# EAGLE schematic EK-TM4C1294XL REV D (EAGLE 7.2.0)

## Sheet 1 of 6: TM4C129ENCPDT GPIO
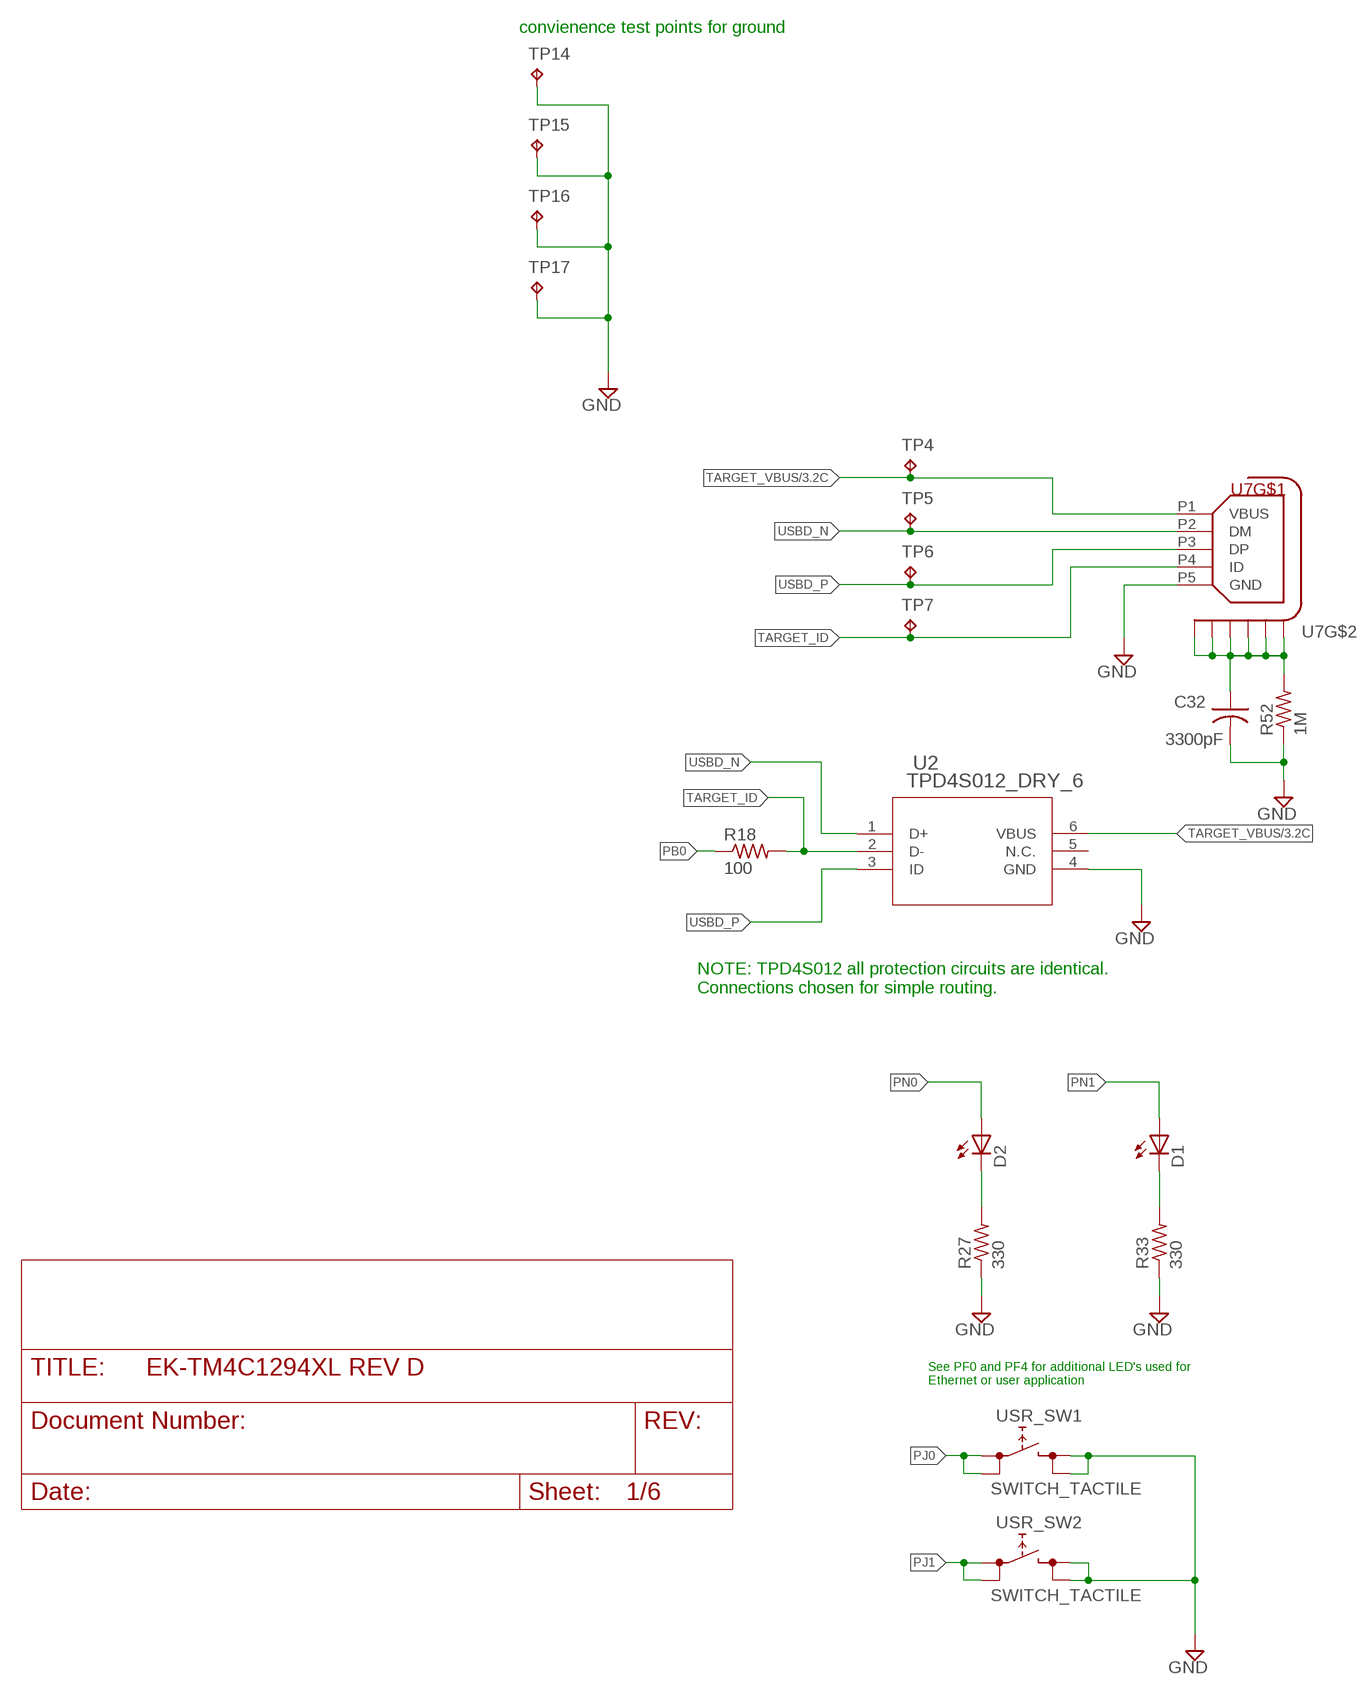
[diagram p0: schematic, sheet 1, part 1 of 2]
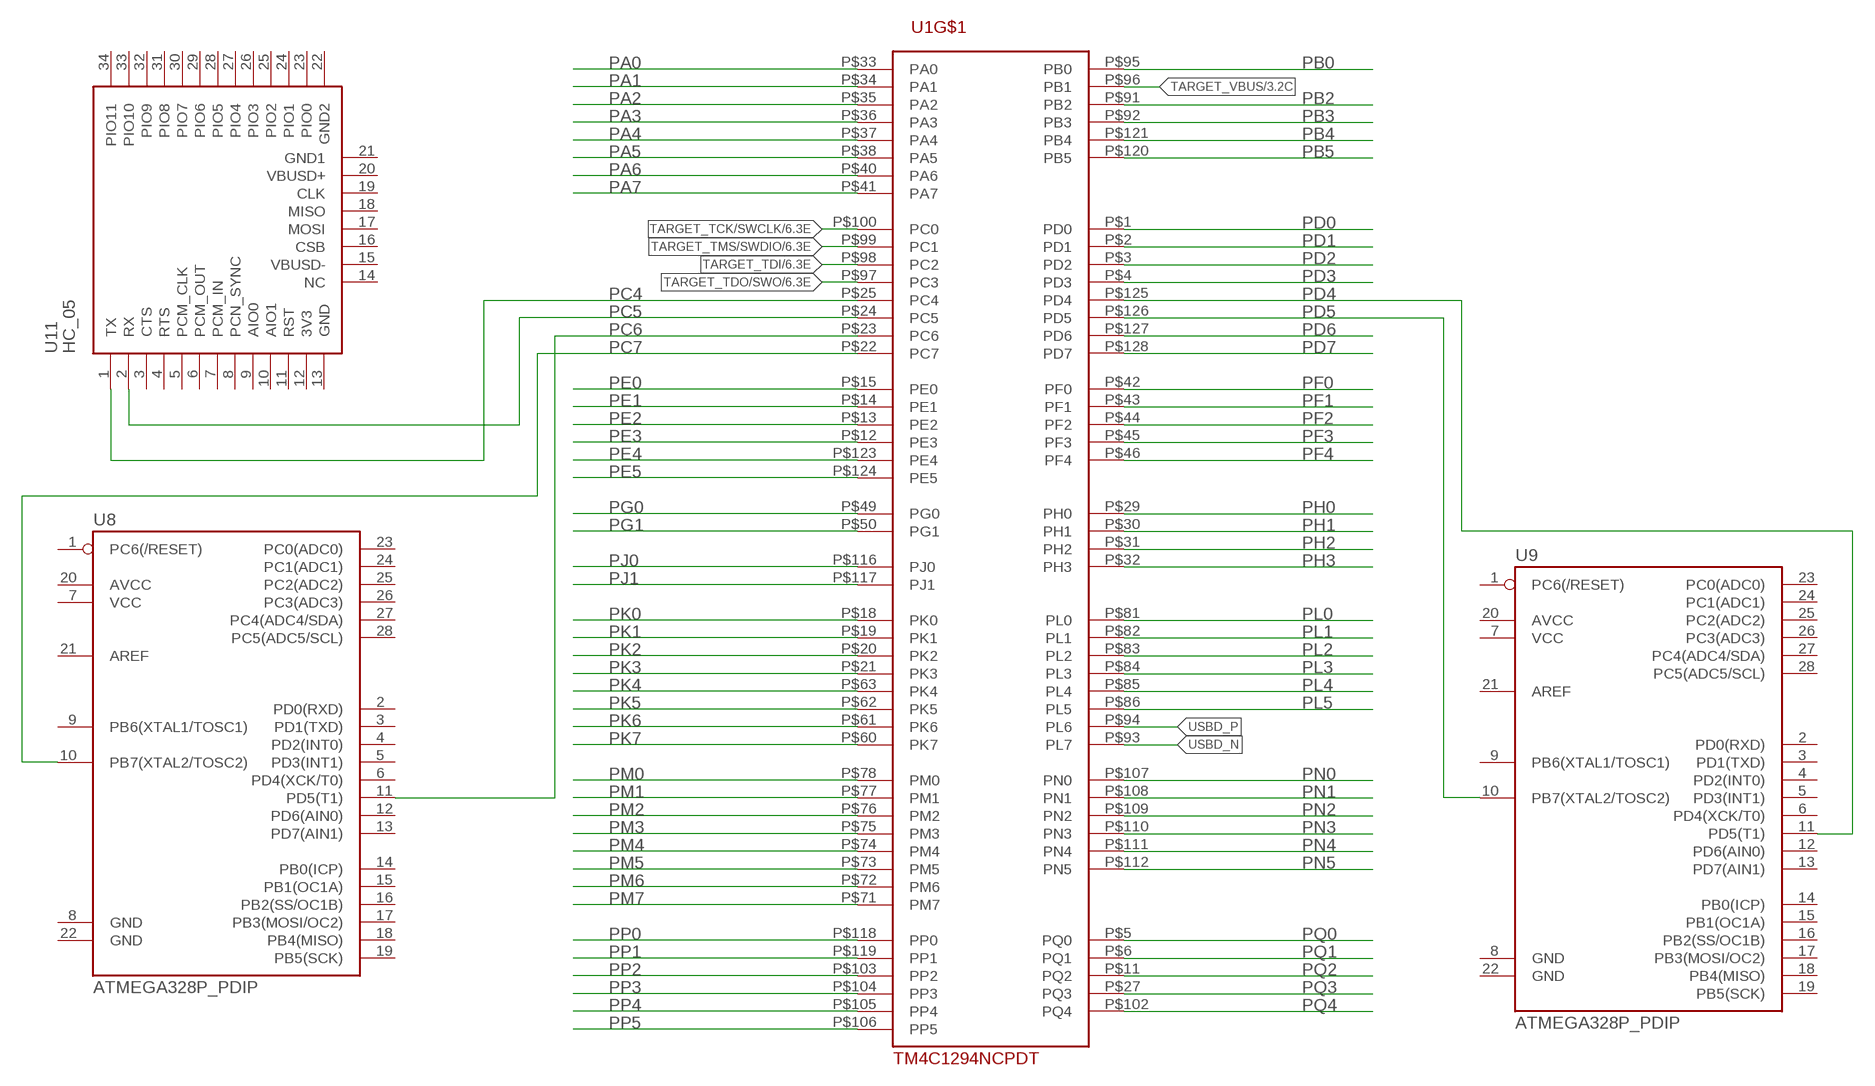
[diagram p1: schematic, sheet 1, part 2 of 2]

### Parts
C32  3300pF  C-USC0603  [C0603]
D1  LEDCHIPLED_0603  [CHIPLED_0603]
D2  LEDCHIPLED_0603  [CHIPLED_0603]
R18  100  R-US_R0402  [R0402]
R27  330  R-US_R0402  [R0402]
R33  330  R-US_R0402  [R0402]
R52  1M  R-US_R0603  [R0603]
TP4  TPPAD1-13  [P1-13]
TP5  TPPAD1-13  [P1-13]
TP6  TPPAD1-13  [P1-13]
TP7  TPPAD1-13  [P1-13]
TP14  TPPAD1-13  [P1-13]
TP15  TPPAD1-13  [P1-13]
TP16  TPPAD1-13  [P1-13]
TP17  TPPAD1-13  [P1-13]
U1  TM4C1294NCPDT  [TQFP-128]
U2  TPD4S012_DRY_6  [DRY6]
U7  CON_USB_HIROSE_MICRO_AB_ZX62D_AB_5P8  [CON_USB_MICRO_AB_HIROSE_ZX62D-AB-5P8]
U8  ATMEGA328P_PDIP  [DIL28-3]
U9  ATMEGA328P_PDIP  [DIL28-3]
U11  HC_05  [BLUETOOTH_SMD]
USR_SW1  SWITCH_TACTILE  [SWITCH_6MM_6MM_TE_CON_SMD]
USR_SW2  SWITCH_TACTILE  [SWITCH_6MM_6MM_TE_CON_SMD]

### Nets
GND: C32.2 R27.1 R33.1 R52.1 TP14.TP TP15.TP TP16.TP TP17.TP U2.4(GND) U7.P5(GND) USR_SW1.P$3 USR_SW1.P$4 USR_SW2.P$3 USR_SW2.P$4 ; also sheet 2,3,4,5,6
N$6: D1.C R33.2
N$8: C32.1 R52.2 U7.P$1(S1) U7.P$2(S2) U7.P$3(S3) U7.P$4(S4) U7.P$5(S5) U7.P$6(S6)
N$14: D2.C R27.2
PA0: U1.P$33(PA0) ; also sheet 2,3
PA1: U1.P$34(PA1) ; also sheet 2,3
PA2: U1.P$35(PA2) ; also sheet 2,3
PA3: U1.P$36(PA3) ; also sheet 2,3
PA4: U1.P$37(PA4) ; also sheet 2,3
PA5: U1.P$38(PA5) ; also sheet 2,3
PA6: U1.P$40(PA6) ; also sheet 2,3
PA7: U1.P$41(PA7) ; also sheet 2,3
PB0: R18.1 U1.P$95(PB0) ; also sheet 3
PB2: U1.P$91(PB2) ; also sheet 2,3
PB3: U1.P$92(PB3) ; also sheet 2,3
PB4: U1.P$121(PB4) ; also sheet 2,3
PB5: U1.P$120(PB5) ; also sheet 2,3
PC4: U1.P$25(PC4) U11.1(TX) ; also sheet 2,3
PC5: U1.P$24(PC5) U11.2(RX) ; also sheet 2,3
PC6: U1.P$23(PC6) U8.11(PD5(T1)) ; also sheet 2,3
PC7: U1.P$22(PC7) U8.10(PB7(XTAL2/TOSC2)) ; also sheet 2,3
PD0: U1.P$1(PD0) ; also sheet 2,3
PD1: U1.P$2(PD1) ; also sheet 2,3
PD2: U1.P$3(PD2) ; also sheet 2,3
PD3: U1.P$4(PD3) ; also sheet 2,3
PD4: U1.P$125(PD4) U9.11(PD5(T1)) ; also sheet 2,3
PD5: U1.P$126(PD5) U9.10(PB7(XTAL2/TOSC2)) ; also sheet 2,3
PD6: U1.P$127(PD6) ; also sheet 3,5
PD7: U1.P$128(PD7) ; also sheet 2,3
PE0: U1.P$15(PE0) ; also sheet 2,3
PE1: U1.P$14(PE1) ; also sheet 2,3
PE2: U1.P$13(PE2) ; also sheet 2,3
PE3: U1.P$12(PE3) ; also sheet 2,3
PE4: U1.P$123(PE4) ; also sheet 2,3
PE5: U1.P$124(PE5) ; also sheet 2,3
PF0: U1.P$42(PF0) ; also sheet 3,4
PF1: U1.P$43(PF1) ; also sheet 2,3
PF2: U1.P$44(PF2) ; also sheet 2,3
PF3: U1.P$45(PF3) ; also sheet 2,3
PF4: U1.P$46(PF4) ; also sheet 3,4
PG0: U1.P$49(PG0) ; also sheet 2,3
PG1: U1.P$50(PG1) ; also sheet 2,3
PH0: U1.P$29(PH0) ; also sheet 2,3
PH1: U1.P$30(PH1) ; also sheet 2,3
PH2: U1.P$31(PH2) ; also sheet 2,3
PH3: U1.P$32(PH3) ; also sheet 2,3
PJ0: U1.P$116(PJ0) USR_SW1.P$1 USR_SW1.P$2 ; also sheet 3
PJ1: U1.P$117(PJ1) USR_SW2.P$1 USR_SW2.P$2 ; also sheet 3
PK0: U1.P$18(PK0) ; also sheet 2,3
PK1: U1.P$19(PK1) ; also sheet 2,3
PK2: U1.P$20(PK2) ; also sheet 2,3
PK3: U1.P$21(PK3) ; also sheet 2,3
PK4: U1.P$63(PK4) ; also sheet 2,3
PK5: U1.P$62(PK5) ; also sheet 2,3
PK6: U1.P$61(PK6) ; also sheet 2,3
PK7: U1.P$60(PK7) ; also sheet 2,3
PL0: U1.P$81(PL0) ; also sheet 2,3
PL1: U1.P$82(PL1) ; also sheet 2,3
PL2: U1.P$83(PL2) ; also sheet 2,3
PL3: U1.P$84(PL3) ; also sheet 2,3
PL4: U1.P$85(PL4) ; also sheet 2,3
PL5: U1.P$86(PL5) ; also sheet 2,3
PM0: U1.P$78(PM0) ; also sheet 2,3
PM1: U1.P$77(PM1) ; also sheet 2,3
PM2: U1.P$76(PM2) ; also sheet 2,3
PM3: U1.P$75(PM3) ; also sheet 2,3
PM4: U1.P$74(PM4) ; also sheet 2,3
PM5: U1.P$73(PM5) ; also sheet 2,3
PM6: U1.P$72(PM6) ; also sheet 2,3
PM7: U1.P$71(PM7) ; also sheet 2,3
PN0: D2.A U1.P$107(PN0) ; also sheet 3
PN1: D1.A U1.P$108(PN1) ; also sheet 3
PN2: U1.P$109(PN2) ; also sheet 2,3
PN3: U1.P$110(PN3) ; also sheet 2,3
PN4: U1.P$111(PN4) ; also sheet 2,3
PN5: U1.P$112(PN5) ; also sheet 2,3
PP0: U1.P$118(PP0) ; also sheet 2,3
PP1: U1.P$119(PP1) ; also sheet 2,3
PP2: U1.P$103(PP2) ; also sheet 2,3
PP3: U1.P$104(PP3) ; also sheet 2,3
PP4: U1.P$105(PP4) ; also sheet 2,3
PP5: U1.P$106(PP5) ; also sheet 2,3
PQ0: U1.P$5(PQ0) ; also sheet 2,3
PQ1: U1.P$6(PQ1) ; also sheet 2,3
PQ2: U1.P$11(PQ2) ; also sheet 2,3
PQ3: U1.P$27(PQ3) ; also sheet 2,3
PQ4: U1.P$102(PQ4) ; also sheet 3,5
TARGET_ID: R18.2 TP7.TP U2.2(D-) U7.P4(ID)
TARGET_TCK/SWCLK: U1.P$100(PC0) ; also sheet 6
TARGET_TDI: U1.P$98(PC2) ; also sheet 6
TARGET_TDO/SWO: U1.P$97(PC3) ; also sheet 6
TARGET_TMS/SWDIO: U1.P$99(PC1) ; also sheet 6
TARGET_VBUS: TP4.TP U1.P$96(PB1) U2.6(VBUS) U7.P1(VBUS) ; also sheet 3,5
USBD_N [USB]: TP5.TP U1.P$93(PL7) U2.1(D+) U7.P2(DM)
USBD_P [USB]: TP6.TP U1.P$94(PL6) U2.3(ID) U7.P3(DP)
Unconnected: U2.5(N.C.) U8.1(PC6(/RESET)) U8.2(PD0(RXD)) U8.3(PD1(TXD)) U8.4(PD2(INT0)) U8.5(PD3(INT1)) U8.6(PD4(XCK/T0)) U8.7(VCC) U8.8(GND) U8.9(PB6(XTAL1/TOSC1)) U8.12(PD6(AIN0)) U8.13(PD7(AIN1)) U8.14(PB0(ICP)) U8.15(PB1(OC1A)) U8.16(PB2(SS/OC1B)) U8.17(PB3(MOSI/OC2)) U8.18(PB4(MISO)) U8.19(PB5(SCK)) U8.20(AVCC) U8.21(AREF) U8.22(GND) U8.23(PC0(ADC0)) U8.24(PC1(ADC1)) U8.25(PC2(ADC2)) U8.26(PC3(ADC3)) U8.27(PC4(ADC4/SDA)) U8.28(PC5(ADC5/SCL)) U9.1(PC6(/RESET)) U9.2(PD0(RXD)) U9.3(PD1(TXD)) U9.4(PD2(INT0)) U9.5(PD3(INT1)) U9.6(PD4(XCK/T0)) U9.7(VCC) U9.8(GND) U9.9(PB6(XTAL1/TOSC1)) U9.12(PD6(AIN0)) U9.13(PD7(AIN1)) U9.14(PB0(ICP)) U9.15(PB1(OC1A)) U9.16(PB2(SS/OC1B)) U9.17(PB3(MOSI/OC2)) U9.18(PB4(MISO)) U9.19(PB5(SCK)) U9.20(AVCC) U9.21(AREF) U9.22(GND) U9.23(PC0(ADC0)) U9.24(PC1(ADC1)) U9.25(PC2(ADC2)) U9.26(PC3(ADC3)) U9.27(PC4(ADC4/SDA)) U9.28(PC5(ADC5/SCL)) U11.3(CTS) U11.4(RTS) U11.5(PCM_CLK) U11.6(PCM_OUT) U11.7(PCM_IN) U11.8(PCN_SYNC) U11.9(AIO0) U11.10(AIO1) U11.11(RST) U11.12(3V3) U11.13(GND) U11.14(NC) U11.15(VBUSD-) U11.16(CSB) U11.17(MOSI) U11.18(MISO) U11.19(CLK) U11.20(VBUSD+) U11.21(GND1) U11.22(GND2) U11.23(PIO0) U11.24(PIO1) U11.25(PIO2) U11.26(PIO3) U11.27(PIO4) U11.28(PIO5) U11.29(PIO6) U11.30(PIO7) U11.31(PIO8) U11.32(PIO9) U11.33(PIO10) U11.34(PIO11)

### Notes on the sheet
- convienence test points for ground
- NOTE: TPD4S012 all protection circuits are identical.  
  Connections chosen for simple routing.
- See PF0 and PF4 for additional LED's used for
  Ethernet or user application

## Sheet 2 of 6: BoosterPack Interface
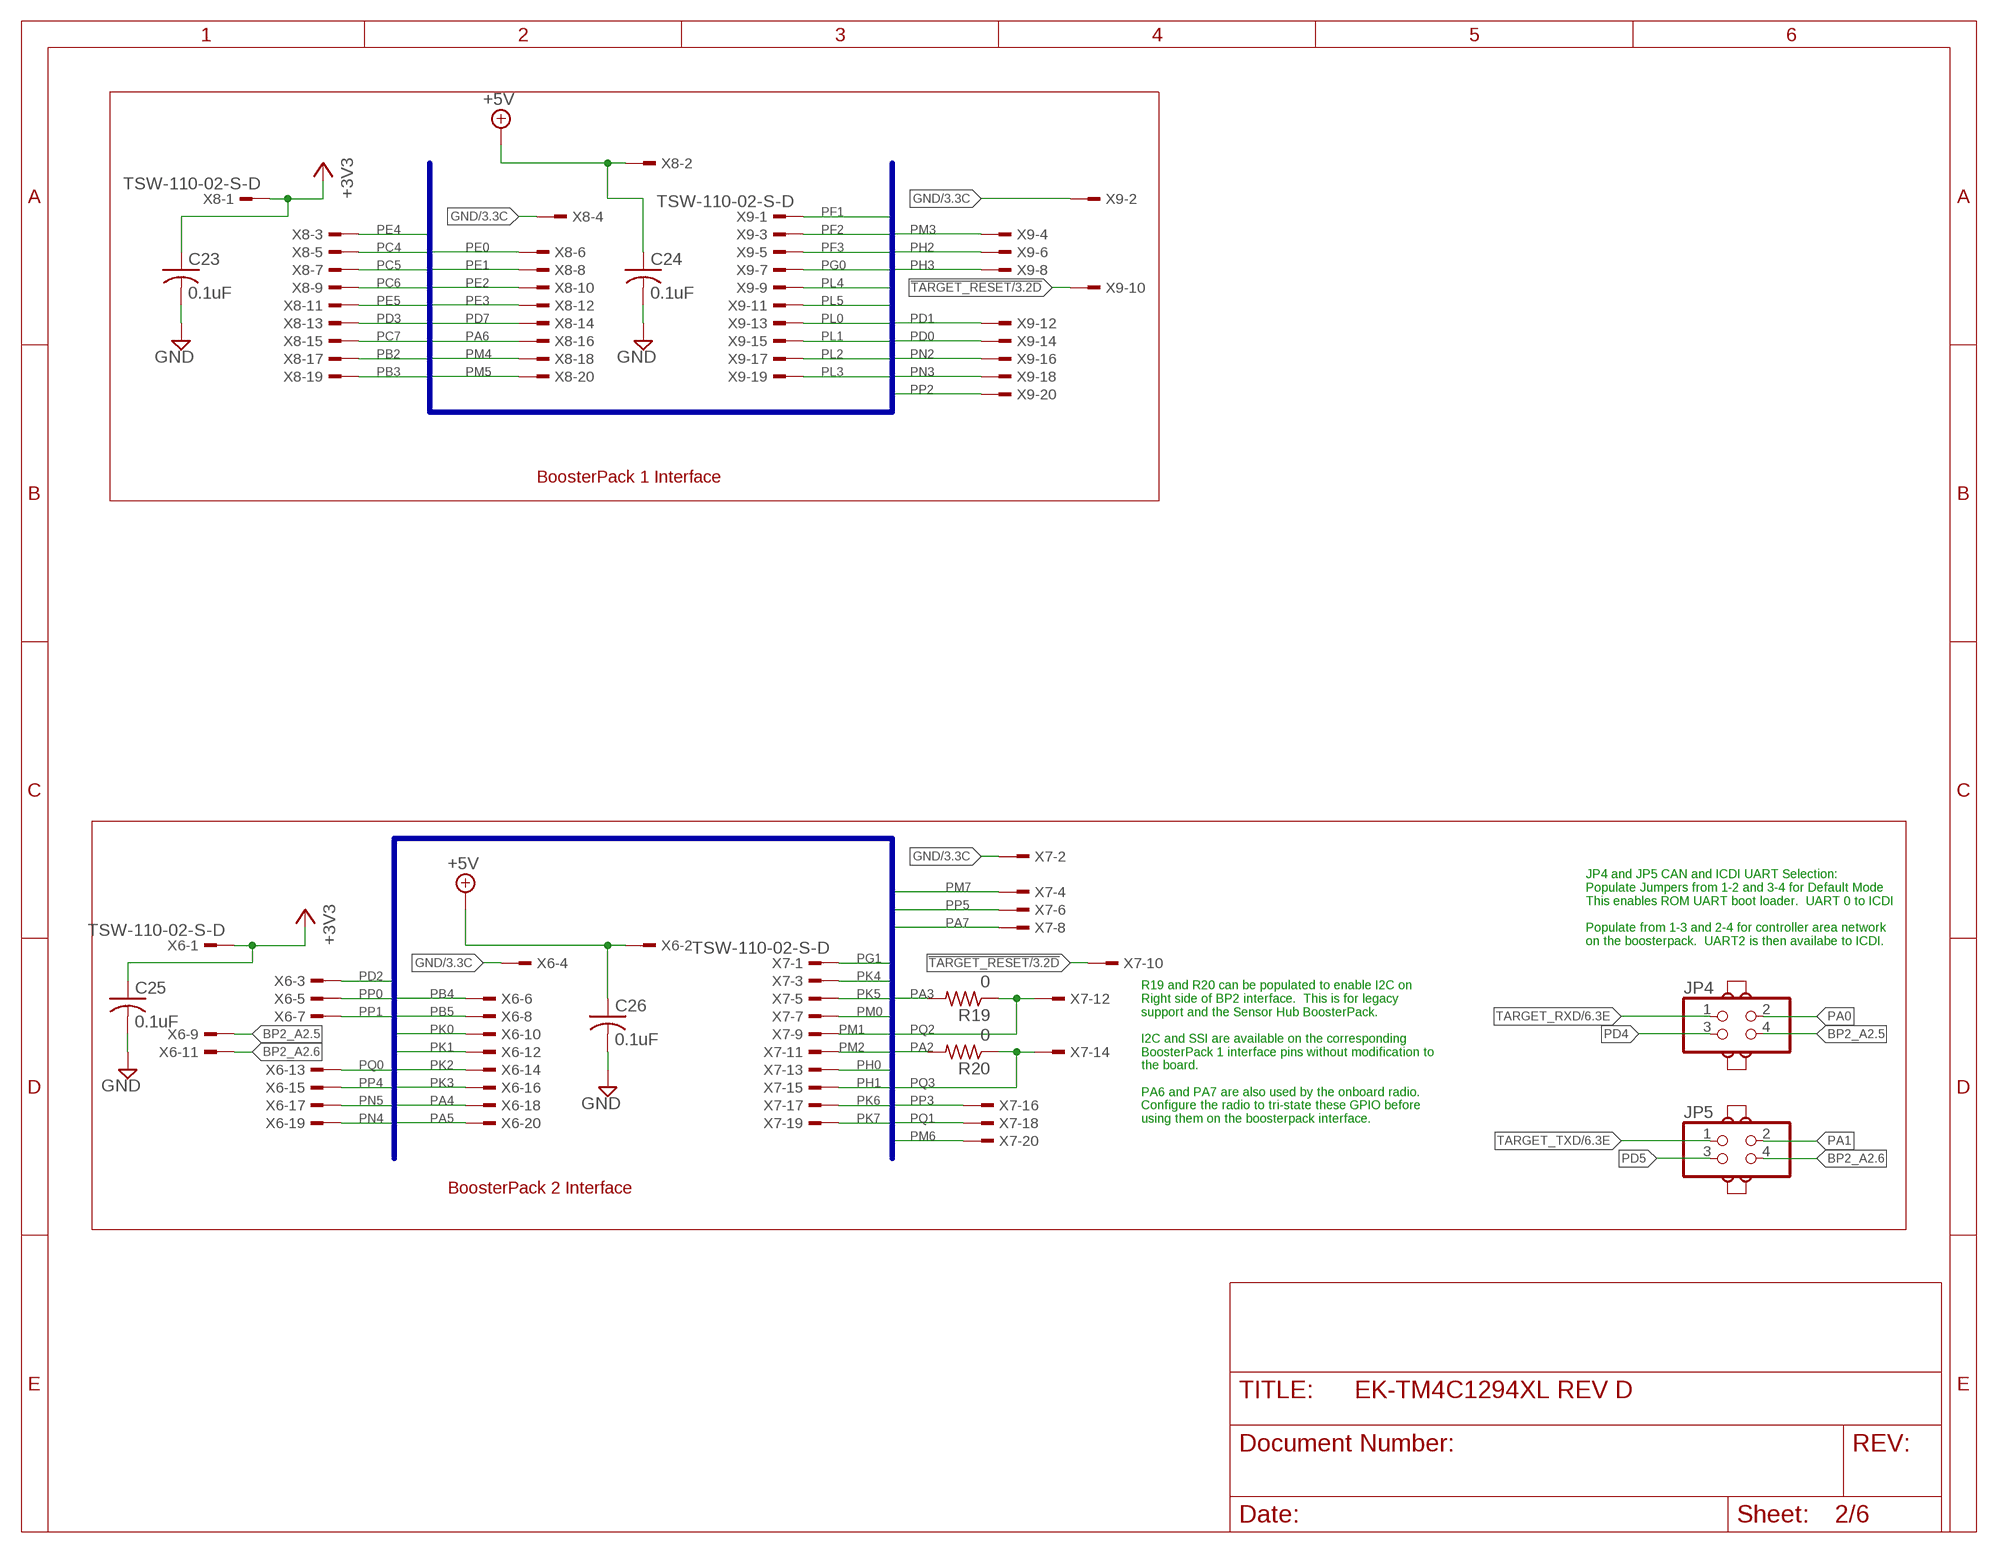
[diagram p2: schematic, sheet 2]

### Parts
C23  0.1uF  C-USC0402  [C0402]
C24  0.1uF  C-USC0402  [C0402]
C25  0.1uF  C-USC0402  [C0402]
C26  0.1uF  C-USC0402  [C0402]
J4  JUMPER  [JUMP]
J5  JUMPER  [JUMP]
J6  JUMPER  [JUMP]
J7  JUMPER  [JUMP]
JP4  PINHD-2X2  [2X02]
JP5  PINHD-2X2  [2X02]
R19  0  R-US_R0402  [R0402]
R20  0  R-US_R0402  [R0402]
X6  TSW-110-02-S-D  [TSW-110-02-S-D]
X7  TSW-110-02-S-D  [TSW-110-02-S-D]
X8  TSW-110-02-S-D  [TSW-110-02-S-D]
X9  TSW-110-02-S-D  [TSW-110-02-S-D]

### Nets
!TARGET_RESET: X7.10 X9.10 ; also sheet 3,5,6
+3V3: C23.1 C25.1 X6.1 X8.1 ; also sheet 3,5,6
+5V: C24.1 C26.1 X6.2 X8.2 ; also sheet 3,5
BP2_A2.5: JP4.4 X6.9
BP2_A2.6: JP5.4 X6.11
GND: C23.2 C24.2 C25.2 C26.2 X6.4 X7.2 X8.4 X9.2 ; also sheet 1,3,4,5,6
PA0: JP4.2 ; also sheet 1,3
PA1: JP5.2 ; also sheet 1,3
PA2: R20.2 ; also sheet 1,3
PA3: R19.2 ; also sheet 1,3
PA4: X6.18 ; also sheet 1,3
PA5: X6.20 ; also sheet 1,3
PA6: X8.16 ; also sheet 1,3
PA7: X7.8 ; also sheet 1,3
PB2: X8.17 ; also sheet 1,3
PB3: X8.19 ; also sheet 1,3
PB4: X6.6 ; also sheet 1,3
PB5: X6.8 ; also sheet 1,3
PC4: X8.5 ; also sheet 1,3
PC5: X8.7 ; also sheet 1,3
PC6: X8.9 ; also sheet 1,3
PC7: X8.15 ; also sheet 1,3
PD0: X9.14 ; also sheet 1,3
PD1: X9.12 ; also sheet 1,3
PD2: X6.3 ; also sheet 1,3
PD3: X8.13 ; also sheet 1,3
PD4: JP4.3 ; also sheet 1,3
PD5: JP5.3 ; also sheet 1,3
PD7: X8.14 ; also sheet 1,3
PE0: X8.6 ; also sheet 1,3
PE1: X8.8 ; also sheet 1,3
PE2: X8.10 ; also sheet 1,3
PE3: X8.12 ; also sheet 1,3
PE4: X8.3 ; also sheet 1,3
PE5: X8.11 ; also sheet 1,3
PF1: X9.1 ; also sheet 1,3
PF2: X9.3 ; also sheet 1,3
PF3: X9.5 ; also sheet 1,3
PG0: X9.7 ; also sheet 1,3
PG1: X7.1 ; also sheet 1,3
PH0: X7.13 ; also sheet 1,3
PH1: X7.15 ; also sheet 1,3
PH2: X9.6 ; also sheet 1,3
PH3: X9.8 ; also sheet 1,3
PK0: X6.10 ; also sheet 1,3
PK1: X6.12 ; also sheet 1,3
PK2: X6.14 ; also sheet 1,3
PK3: X6.16 ; also sheet 1,3
PK4: X7.3 ; also sheet 1,3
PK5: X7.5 ; also sheet 1,3
PK6: X7.17 ; also sheet 1,3
PK7: X7.19 ; also sheet 1,3
PL0: X9.13 ; also sheet 1,3
PL1: X9.15 ; also sheet 1,3
PL2: X9.17 ; also sheet 1,3
PL3: X9.19 ; also sheet 1,3
PL4: X9.9 ; also sheet 1,3
PL5: X9.11 ; also sheet 1,3
PM0: X7.7 ; also sheet 1,3
PM1: X7.9 ; also sheet 1,3
PM2: X7.11 ; also sheet 1,3
PM3: X9.4 ; also sheet 1,3
PM4: X8.18 ; also sheet 1,3
PM5: X8.20 ; also sheet 1,3
PM6: X7.20 ; also sheet 1,3
PM7: X7.4 ; also sheet 1,3
PN2: X9.16 ; also sheet 1,3
PN3: X9.18 ; also sheet 1,3
PN4: X6.19 ; also sheet 1,3
PN5: X6.17 ; also sheet 1,3
PP0: X6.5 ; also sheet 1,3
PP1: X6.7 ; also sheet 1,3
PP2: X9.20 ; also sheet 1,3
PP3: X7.16 ; also sheet 1,3
PP4: X6.15 ; also sheet 1,3
PP5: X7.6 ; also sheet 1,3
PQ0: X6.13 ; also sheet 1,3
PQ1: X7.18 ; also sheet 1,3
PQ2: R19.1 X7.12 ; also sheet 1,3
PQ3: R20.1 X7.14 ; also sheet 1,3
TARGET_RXD: JP4.1 ; also sheet 6
TARGET_TXD: JP5.1 ; also sheet 6

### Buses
GPIO:PA[0..7],PB[0..5],PC[0..7],PD[0..7],PE[0..5],PF[0..4],PG[0..1],PH[0..3],PJ[0..1],PK[0..7],PL[0..7],PM[0..7],PN[0..5],PP[0..5],PQ[0..4]

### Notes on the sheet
- BoosterPack 1 Interface
- JP4 and JP5 CAN and ICDI UART Selection:
  Populate Jumpers from 1-2 and 3-4 for Default Mode
  This enables ROM UART boot loader.  UART 0 to ICDI
  
  Populate from 1-3 and 2-4 for controller area network
  on the boosterpack.  UART2 is then availabe to ICDI.
- R19 and R20 can be populated to enable I2C on 
  Right side of BP2 interface.  This is for legacy 
  support and the Sensor Hub BoosterPack.
  
  I2C and SSI are available on the corresponding
  BoosterPack 1 interface pins without modification to
  the board.
  
  PA6 and PA7 are also used by the onboard radio. 
  Configure the radio to tri-state these GPIO before 
  using them on the boosterpack interface.
- BoosterPack 2 Interface

## Sheet 3 of 6: GPIO Breakout
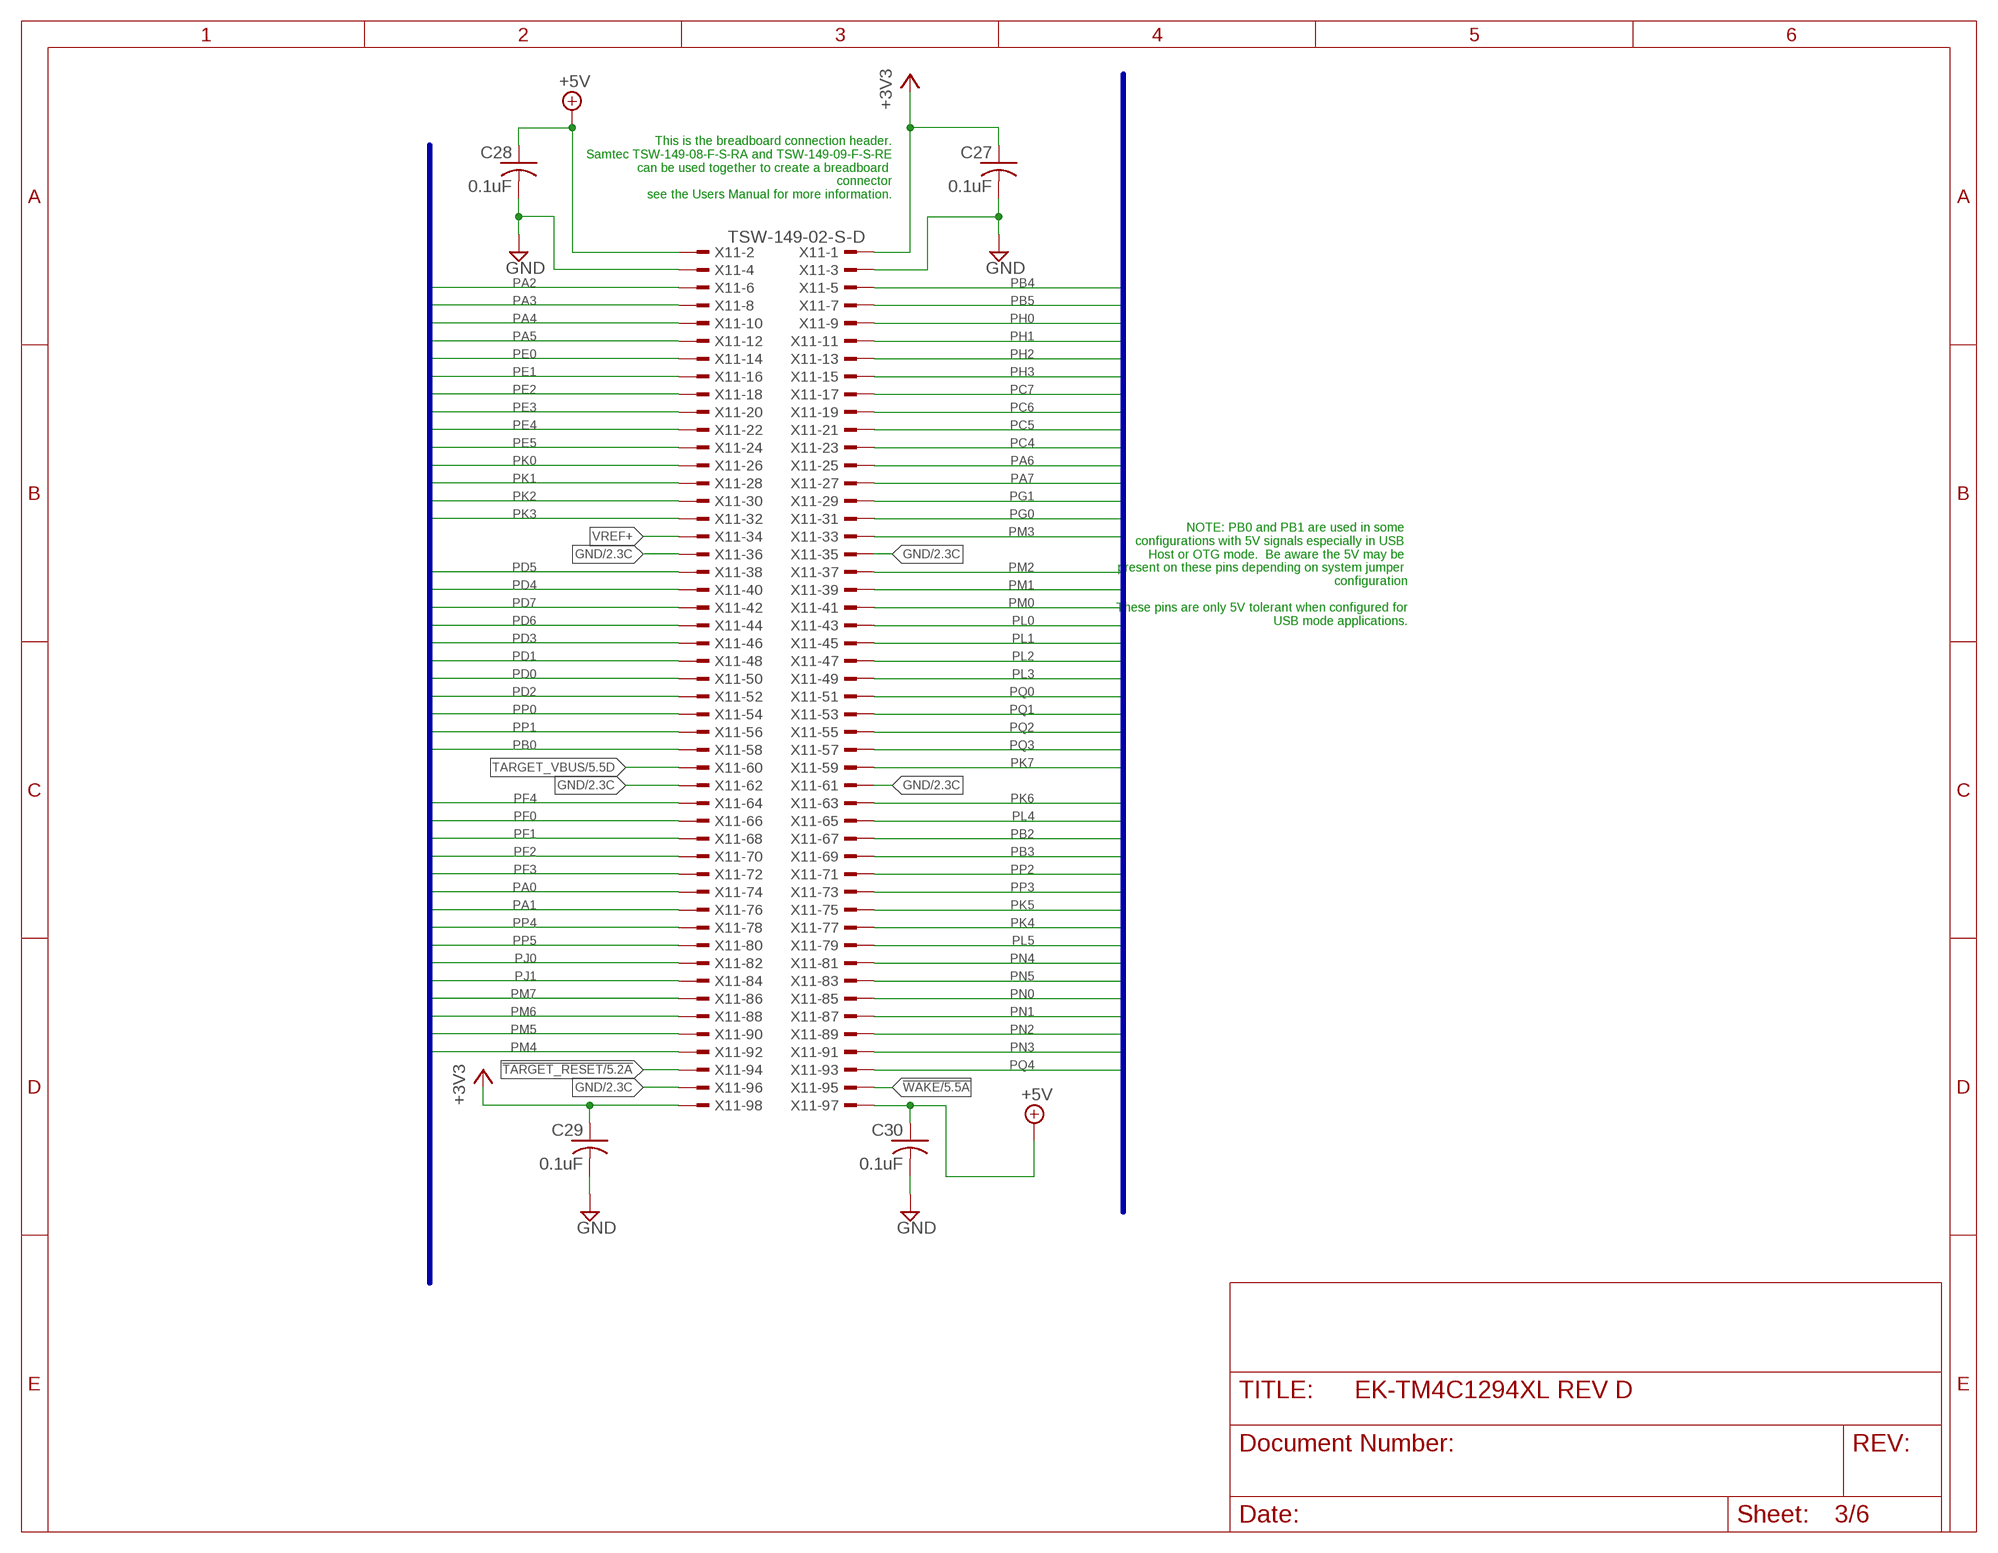
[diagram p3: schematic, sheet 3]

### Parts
C27  0.1uF  C-USC0402  [C0402]
C28  0.1uF  C-USC0402  [C0402]
C29  0.1uF  C-USC0402  [C0402]
C30  0.1uF  C-USC0402  [C0402]
X11  TSW-149-02-S-D  [TSW-149-02-S-D]

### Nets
!TARGET_RESET: X11.94 ; also sheet 2,5,6
!WAKE: X11.95 ; also sheet 5
+3V3: C27.1 C29.1 X11.1 X11.98 ; also sheet 2,5,6
+5V: C28.1 C30.1 X11.2 X11.97 ; also sheet 2,5
GND: C27.2 C28.2 C29.2 C30.2 X11.3 X11.4 X11.35 X11.36 X11.61 X11.62 X11.96 ; also sheet 1,2,4,5,6
PA0: X11.74 ; also sheet 1,2
PA1: X11.76 ; also sheet 1,2
PA2: X11.6 ; also sheet 1,2
PA3: X11.8 ; also sheet 1,2
PA4: X11.10 ; also sheet 1,2
PA5: X11.12 ; also sheet 1,2
PA6: X11.25 ; also sheet 1,2
PA7: X11.27 ; also sheet 1,2
PB0: X11.58 ; also sheet 1
PB2: X11.67 ; also sheet 1,2
PB3: X11.69 ; also sheet 1,2
PB4: X11.5 ; also sheet 1,2
PB5: X11.7 ; also sheet 1,2
PC4: X11.23 ; also sheet 1,2
PC5: X11.21 ; also sheet 1,2
PC6: X11.19 ; also sheet 1,2
PC7: X11.17 ; also sheet 1,2
PD0: X11.50 ; also sheet 1,2
PD1: X11.48 ; also sheet 1,2
PD2: X11.52 ; also sheet 1,2
PD3: X11.46 ; also sheet 1,2
PD4: X11.40 ; also sheet 1,2
PD5: X11.38 ; also sheet 1,2
PD6: X11.44 ; also sheet 1,5
PD7: X11.42 ; also sheet 1,2
PE0: X11.14 ; also sheet 1,2
PE1: X11.16 ; also sheet 1,2
PE2: X11.18 ; also sheet 1,2
PE3: X11.20 ; also sheet 1,2
PE4: X11.22 ; also sheet 1,2
PE5: X11.24 ; also sheet 1,2
PF0: X11.66 ; also sheet 1,4
PF1: X11.68 ; also sheet 1,2
PF2: X11.70 ; also sheet 1,2
PF3: X11.72 ; also sheet 1,2
PF4: X11.64 ; also sheet 1,4
PG0: X11.31 ; also sheet 1,2
PG1: X11.29 ; also sheet 1,2
PH0: X11.9 ; also sheet 1,2
PH1: X11.11 ; also sheet 1,2
PH2: X11.13 ; also sheet 1,2
PH3: X11.15 ; also sheet 1,2
PJ0: X11.82 ; also sheet 1
PJ1: X11.84 ; also sheet 1
PK0: X11.26 ; also sheet 1,2
PK1: X11.28 ; also sheet 1,2
PK2: X11.30 ; also sheet 1,2
PK3: X11.32 ; also sheet 1,2
PK4: X11.77 ; also sheet 1,2
PK5: X11.75 ; also sheet 1,2
PK6: X11.63 ; also sheet 1,2
PK7: X11.59 ; also sheet 1,2
PL0: X11.43 ; also sheet 1,2
PL1: X11.45 ; also sheet 1,2
PL2: X11.47 ; also sheet 1,2
PL3: X11.49 ; also sheet 1,2
PL4: X11.65 ; also sheet 1,2
PL5: X11.79 ; also sheet 1,2
PM0: X11.41 ; also sheet 1,2
PM1: X11.39 ; also sheet 1,2
PM2: X11.37 ; also sheet 1,2
PM3: X11.33 ; also sheet 1,2
PM4: X11.92 ; also sheet 1,2
PM5: X11.90 ; also sheet 1,2
PM6: X11.88 ; also sheet 1,2
PM7: X11.86 ; also sheet 1,2
PN0: X11.85 ; also sheet 1
PN1: X11.87 ; also sheet 1
PN2: X11.89 ; also sheet 1,2
PN3: X11.91 ; also sheet 1,2
PN4: X11.81 ; also sheet 1,2
PN5: X11.83 ; also sheet 1,2
PP0: X11.54 ; also sheet 1,2
PP1: X11.56 ; also sheet 1,2
PP2: X11.71 ; also sheet 1,2
PP3: X11.73 ; also sheet 1,2
PP4: X11.78 ; also sheet 1,2
PP5: X11.80 ; also sheet 1,2
PQ0: X11.51 ; also sheet 1,2
PQ1: X11.53 ; also sheet 1,2
PQ2: X11.55 ; also sheet 1,2
PQ3: X11.57 ; also sheet 1,2
PQ4: X11.93 ; also sheet 1,5
TARGET_VBUS: X11.60 ; also sheet 1,5
VREF+: X11.34 ; also sheet 5

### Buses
GPIO:PA[0..7],PB[0..5],PC[0..7],PD[0..7],PE[0..5],PF[0..4],PG[0..1],PH[0..3],PJ[0..1],PK[0..7],PL[0..7],PM[0..7],PN[0..5],PP[0..5],PQ[0..4]

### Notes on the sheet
- This is the breadboard connection header.
  Samtec TSW-149-08-F-S-RA and TSW-149-09-F-S-RE
  can be used together to create a breadboard 
  connector
  see the Users Manual for more information.
- NOTE: PB0 and PB1 are used in some 
  configurations with 5V signals especially in USB 
  Host or OTG mode.  Be aware the 5V may be 
  present on these pins depending on system jumper 
  configuration
  
  These pins are only 5V tolerant when configured for
  USB mode applications.

## Sheet 4 of 6: Ethernet
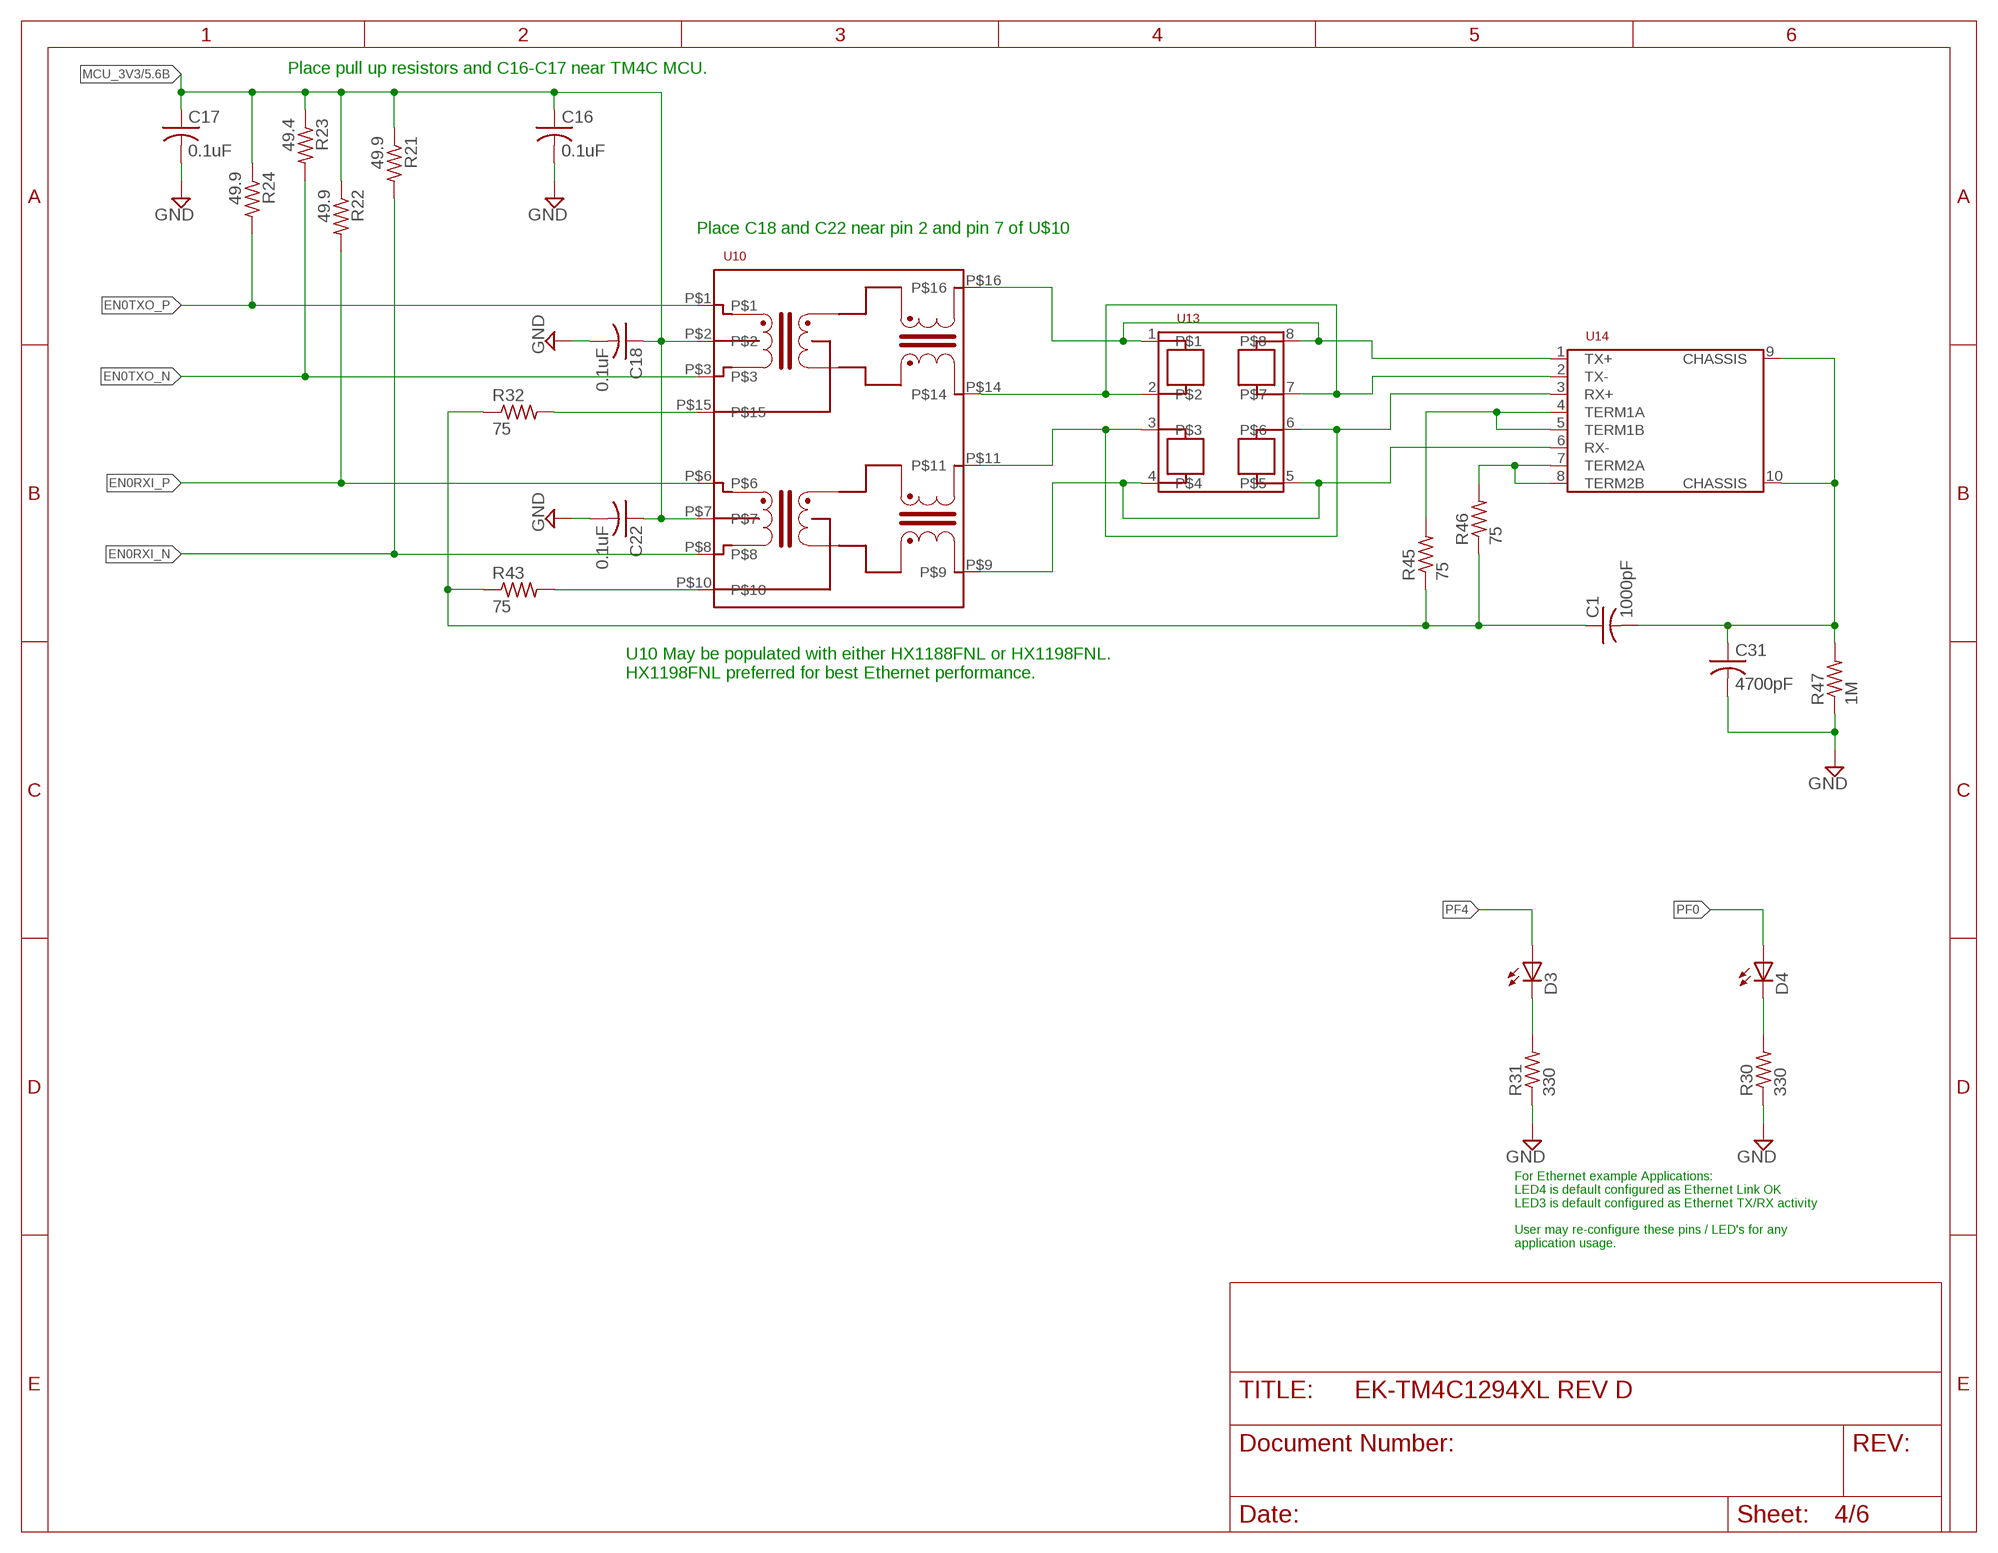
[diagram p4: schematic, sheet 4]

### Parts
C1  1000pF  C-USC1210  [C1210]
C16  0.1uF  C-USC0402  [C0402]
C17  0.1uF  C-USC0402  [C0402]
C18  0.1uF  C-USC0402  [C0402]
C22  0.1uF  C-USC0402  [C0402]
C31  4700pF  C-USC1812  [C1812]
D3  LEDCHIPLED_0603  [CHIPLED_0603]
D4  LEDCHIPLED_0603  [CHIPLED_0603]
R21  49.9  R-US_R0402  [R0402]
R22  49.9  R-US_R0402  [R0402]
R23  49.4  R-US_R0402  [R0402]
R24  49.9  R-US_R0402  [R0402]
R30  330  R-US_R0402  [R0402]
R31  330  R-US_R0402  [R0402]
R32  75  R-US_R0402  [R0402]
R43  75  R-US_R0402  [R0402]
R45  75  R-US_R0402  [R0402]
R46  75  R-US_R0402  [R0402]
R47  1M  R-US_R1206  [R1206]
U10  MAG_PULSE_HX1188FNL  [MAG_PULSE_HX1188FNL]
U13  SLVU2.8-4  [D8]
U14  JACK_RJ45_NOMAG_NOLED_TECON  [RJ45_TE_CON_NOMAG_NOLED]

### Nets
CHASSIS: C1.2 C31.1 R47.2 U14.9(CHASSIS) U14.10(CHASSIS)
EN0RXI_N [Ethernet]: R21.2 U10.P$8 ; also sheet 5
EN0RXI_P [Ethernet]: R22.2 U10.P$6 ; also sheet 5
EN0TXO_N [Ethernet]: R23.2 U10.P$3 ; also sheet 5
EN0TXO_P [Ethernet]: R24.2 U10.P$1 ; also sheet 5
GND: C16.2 C17.2 C18.2 C22.2 C31.2 R30.1 R31.1 R47.1 ; also sheet 1,2,3,5,6
JACK_RX_N [Ethernet]: U10.P$9 U13.4 U13.5 U14.6(RX-)
JACK_RX_P [Ethernet]: U10.P$11 U13.3 U13.6 U14.3(RX+)
JACK_TX_N [Ethernet]: U10.P$14 U13.2 U13.7 U14.2(TX-)
JACK_TX_P [Ethernet]: U10.P$16 U13.1 U13.8 U14.1(TX+)
MCU_3V3: C16.1 C17.1 C18.1 C22.1 R21.1 R22.1 R23.1 R24.1 U10.P$2 U10.P$7 ; also sheet 5,6
N$4: D4.C R30.2
N$5: D3.C R31.2
N$32: R32.2 U10.P$15
N$34: R43.2 U10.P$10
N$36: C1.1 R32.1 R43.1 R45.1 R46.1
N$44: R45.2 U14.4(TERM1A) U14.5(TERM1B)
N$45: R46.2 U14.7(TERM2A) U14.8(TERM2B)
PF0: D4.A ; also sheet 1,3
PF4: D3.A ; also sheet 1,3

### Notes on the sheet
- Place pull up resistors and C16-C17 near TM4C MCU.
- Place C18 and C22 near pin 2 and pin 7 of U$10
- U10 May be populated with either HX1188FNL or HX1198FNL. 
  HX1198FNL preferred for best Ethernet performance.
- For Ethernet example Applications: 
  LED4 is default configured as Ethernet Link OK
  LED3 is default configured as Ethernet TX/RX activity
  
  User may re-configure these pins / LED's for any
  application usage.

## Sheet 5 of 6: Power
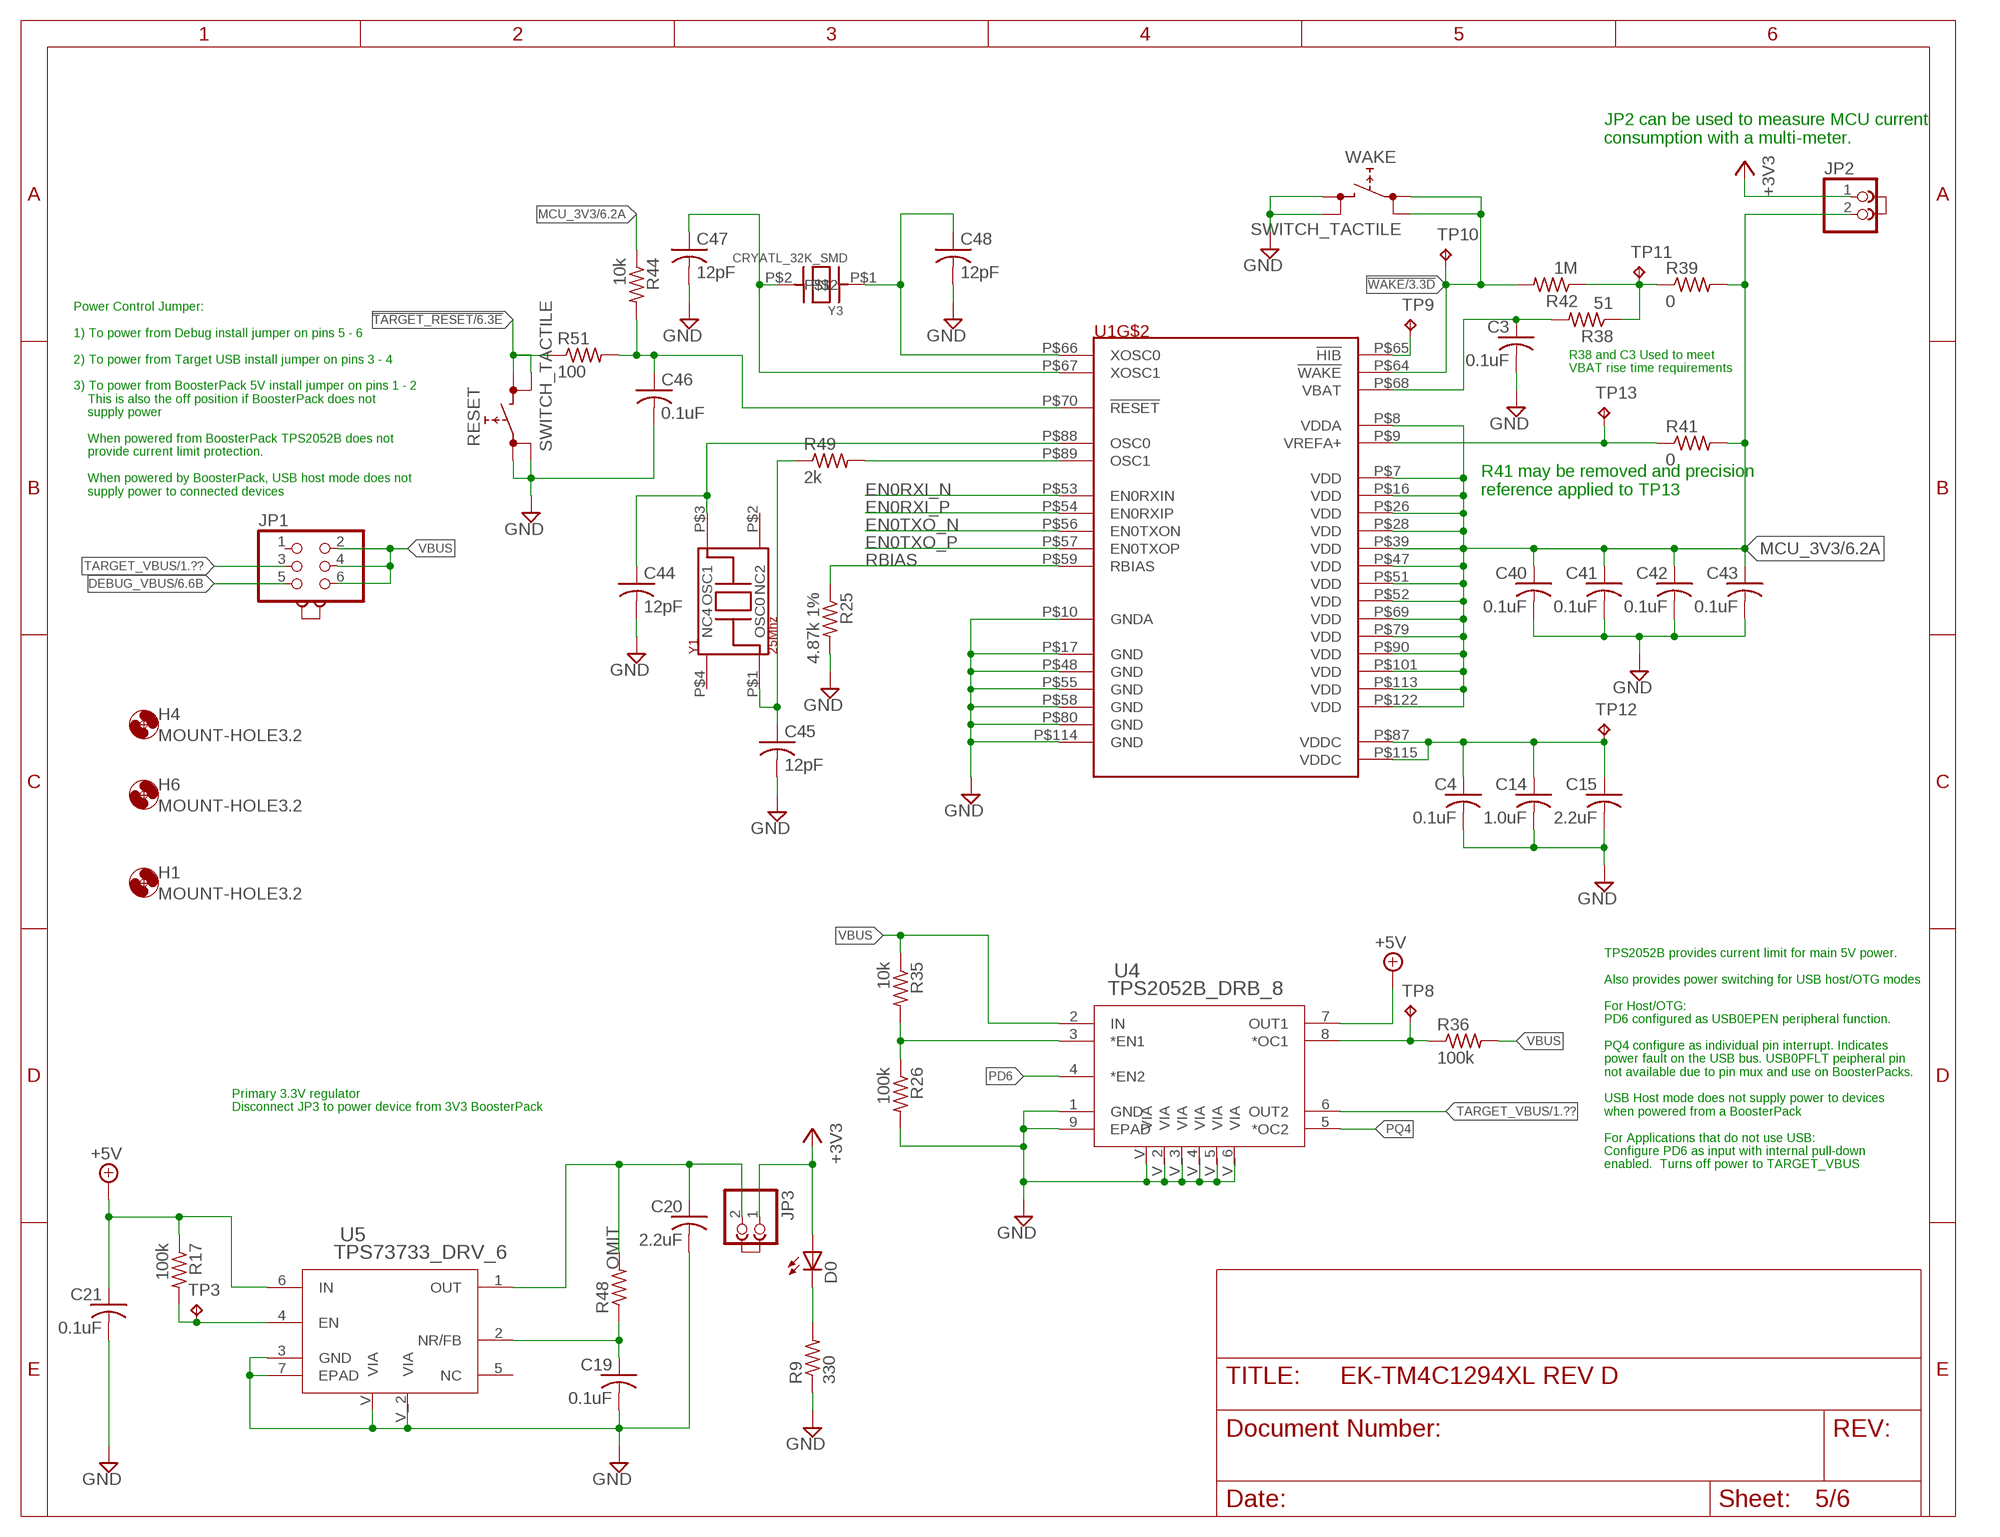
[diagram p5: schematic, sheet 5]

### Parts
C3  0.1uF  C-USC0402  [C0402]
C4  0.1uF  C-USC0402  [C0402]
C14  1.0uF  C-USC0402  [C0402]
C15  2.2uF  C-USC0603K  [C0603K]
C19  0.1uF  C-USC0402  [C0402]
C20  2.2uF  C-USC0603K  [C0603K]
C21  0.1uF  C-USC0402  [C0402]
C40  0.1uF  C-USC0402  [C0402]
C41  0.1uF  C-USC0402  [C0402]
C42  0.1uF  C-USC0402  [C0402]
C43  0.1uF  C-USC0402  [C0402]
C44  12pF  C-USC0402  [C0402]
C45  12pF  C-USC0402  [C0402]
C46  0.1uF  C-USC0402  [C0402]
C47  12pF  C-USC0402  [C0402]
C48  12pF  C-USC0402  [C0402]
D0  LEDCHIPLED_0603  [CHIPLED_0603]
H1  MOUNT-HOLE3.2  [3,2]
H4  MOUNT-HOLE3.2  [3,2]
H6  MOUNT-HOLE3.2  [3,2]
J1  JUMPER  [JUMP]
J2  JUMPER  [JUMP]
J3  JUMPER  [JUMP]
JP1  PINHD-2X3  [2X03]
JP2  PINHD-1X2  [1X02]
JP3  PINHD-1X2  [1X02]
R9  330  R-US_R0402  [R0402]
R17  100k  R-US_R0402  [R0402]
R25  4.87k 1%  R-US_R0402  [R0402]
R26  100k  R-US_R0402  [R0402]
R35  10k  R-US_R0402  [R0402]
R36  100k  R-US_R0402  [R0402]
R38  51  R-US_R0402  [R0402]
R39  0  R-US_R0402  [R0402]
R41  0  R-US_R0402  [R0402]
R42  1M  R-US_R0402  [R0402]
R44  10k  R-US_R0402  [R0402]
R48  R-US_R0402  [R0402]
R49  2k  R-US_R0402  [R0402]
R51  100  R-US_R0402  [R0402]
RESET  SWITCH_TACTILE  [SWITCH_6MM_6MM_TE_CON_SMD]
TP3  TPPAD1-13  [P1-13]
TP8  TPPAD1-13  [P1-13]
TP9  TPPAD1-13  [P1-13]
TP10  TPPAD1-13  [P1-13]
TP11  TPPAD1-13  [P1-13]
TP12  TPPAD1-13  [P1-13]
TP13  TPPAD1-13  [P1-13]
U4  TPS2052B_DRB_8  [DRB8_2P4X1P65]
U5  TPS73733_DRV_6  [DRV6_1P6X1]
WAKE  SWITCH_TACTILE  [SWITCH_6MM_6MM_TE_CON_SMD]
Y1  25Mhz  NX3225GA  [NDK3.2X2.5]
Y3  CRYATL_32K_SMD  [CRYSTAL_32K_SMD]

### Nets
!HIB: TP9.TP U1.P$65(!HIB)
!TARGET_RESET: R51.1 RESET.P$3 RESET.P$4 ; also sheet 2,3,6
!TARGET_RESET_FILTERED: C46.1 R44.2 R51.2 U1.P$70(!RESET)
!WAKE: R42.2 TP10.TP U1.P$64(!WAKE) WAKE.P$1 WAKE.P$2 ; also sheet 3
+3V3: D0.A JP2.1 JP3.1 ; also sheet 2,3,6
+5V: C21.1 R17.1 U4.7(OUT1) U5.6(IN) ; also sheet 2,3
DEBUG_VBUS: JP1.5 ; also sheet 6
EN0RXI_N [Ethernet]: U1.P$53(EN0RXIN) ; also sheet 4
EN0RXI_P [Ethernet]: U1.P$54(EN0RXIP) ; also sheet 4
EN0TXO_N [Ethernet]: U1.P$56(EN0TXON) ; also sheet 4
EN0TXO_P [Ethernet]: U1.P$57(EN0TXOP) ; also sheet 4
GND: C3.2 C4.2 C14.2 C15.2 C19.2 C20.2 C21.2 C40.2 C41.2 C42.2 C43.2 C44.2 C45.2 C46.2 C47.2 C48.2 R9.1 R25.2 R26.2 RESET.P$1 RESET.P$2 U1.P$10(GNDA) U1.P$17(GND) U1.P$48(GND) U1.P$55(GND) U1.P$58(GND) U1.P$80(GND) U1.P$114(GND) U4.1(GND) U4.9(EPAD) U4.V(VIA) U4.V_2(VIA) U4.V_3(VIA) U4.V_4(VIA) U4.V_5(VIA) U4.V_6(VIA) U5.3(GND) U5.7(EPAD) U5.V(VIA) U5.V_2(VIA) WAKE.P$3 WAKE.P$4 ; also sheet 1,2,3,4,6
MCU_3V3: C40.1 C41.1 C42.1 C43.1 JP2.2 R39.2 R41.2 R44.1 U1.P$7(VDD) U1.P$8(VDDA) U1.P$16(VDD) U1.P$26(VDD) U1.P$28(VDD) U1.P$39(VDD) U1.P$47(VDD) U1.P$51(VDD) U1.P$52(VDD) U1.P$69(VDD) U1.P$79(VDD) U1.P$90(VDD) U1.P$101(VDD) U1.P$113(VDD) U1.P$122(VDD) ; also sheet 4,6
N$3: D0.C R9.2
N$7: R26.1 R35.2 U4.3(*EN1)
N$9: C19.1 R48.1 U5.2(NR/FB)
N$10: R36.1 TP8.TP U4.8(*OC1)
N$11: C3.1 R38.2 U1.P$68(VBAT)
N$13: C20.1 JP3.2 R48.2 U5.1(OUT)
N$16: R49.2 U1.P$89(OSC1)
N$29: C45.1 R49.1 Y1.P$1(OSC0)
N$30: C47.1 U1.P$67(XOSC1) Y3.P$2
N$31: C44.1 U1.P$88(OSC0) Y1.P$3(OSC1)
N$33: C48.1 U1.P$66(XOSC0) Y3.P$1
PD6: U4.4(*EN2) ; also sheet 1,3
PQ4: U4.5(*OC2) ; also sheet 1,3
RBIAS: R25.1 U1.P$59(RBIAS)
TARGET_VBUS: JP1.3 U4.6(OUT2) ; also sheet 1,3
TARGET_VDDC: C4.1 C14.1 C15.1 TP12.TP U1.P$87(VDDC) U1.P$115(VDDC)
VBAT: R38.1 R39.1 R42.1 TP11.TP
VBUS: JP1.2 JP1.4 JP1.6 R35.1 R36.2 U4.2(IN)
VREF+: R41.1 TP13.TP U1.P$9(VREFA+) ; also sheet 3
VREG_EN: R17.2 TP3.TP U5.4(EN)
Unconnected: JP1.1 U5.5(NC) Y1.P$2(NC2) Y1.P$4(NC4)

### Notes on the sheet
- JP2 can be used to measure MCU current 
  consumption with a multi-meter.
- R38 and C3 Used to meet 
  VBAT rise time requirements
- Power Control Jumper:
  
  1) To power from Debug install jumper on pins 5 - 6
  
  2) To power from Target USB install jumper on pins 3 - 4
  
  3) To power from BoosterPack 5V install jumper on pins 1 - 2
      This is also the off position if BoosterPack does not 
      supply power
  
      When powered from BoosterPack TPS2052B does not 
      provide current limit protection.
     
      When powered by BoosterPack, USB host mode does not 
      supply power to connected devices
- R41 may be removed and precision
  reference applied to TP13
- Primary 3.3V regulator
  Disconnect JP3 to power device from 3V3 BoosterPack
- TPS2052B provides current limit for main 5V power.
  
  Also provides power switching for USB host/OTG modes
  
  For Host/OTG: 
  PD6 configured as USB0EPEN peripheral function.
  
  PQ4 configure as individual pin interrupt. Indicates 
  power fault on the USB bus. USB0PFLT peipheral pin 
  not available due to pin mux and use on BoosterPacks.
  
  USB Host mode does not supply power to devices
  when powered from a BoosterPack
  
  For Applications that do not use USB:
  Configure PD6 as input with internal pull-down 
  enabled.  Turns off power to TARGET_VBUS

## Sheet 6 of 6: In Circuit Debug
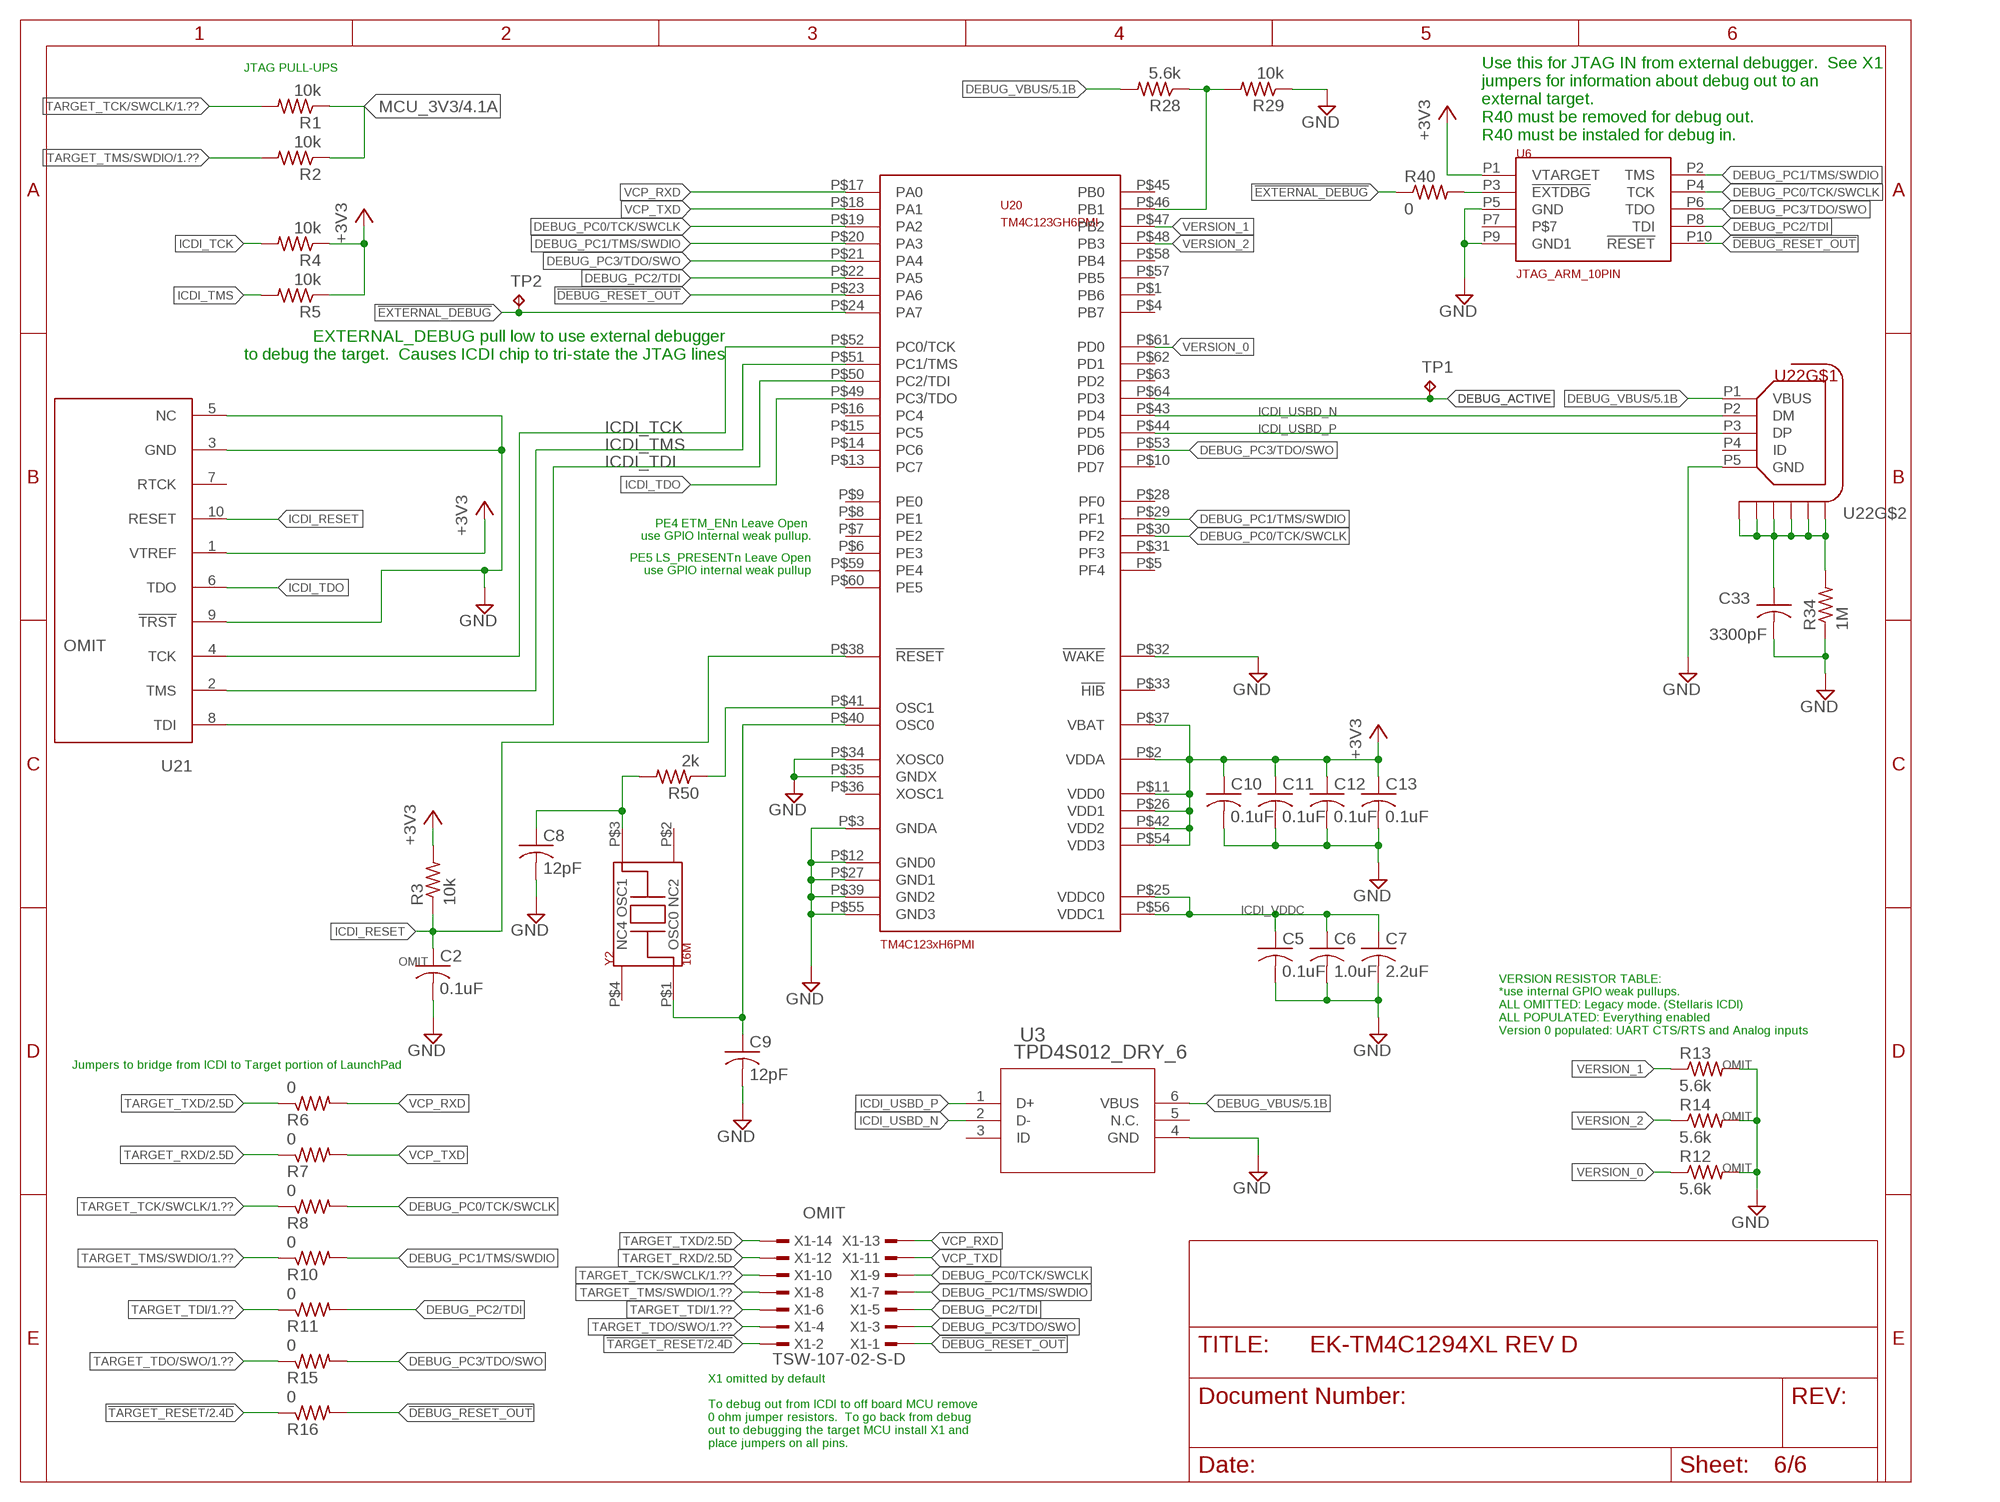
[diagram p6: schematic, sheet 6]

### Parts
C2  0.1uF  C-USC0402  [C0402]
C5  0.1uF  C-USC0402  [C0402]
C6  1.0uF  C-USC0402  [C0402]
C7  2.2uF  C-USC0603  [C0603]
C8  12pF  C-USC0402  [C0402]
C9  12pF  C-USC0402  [C0402]
C10  0.1uF  C-USC0402  [C0402]
C11  0.1uF  C-USC0402  [C0402]
C12  0.1uF  C-USC0402  [C0402]
C13  0.1uF  C-USC0402  [C0402]
C33  3300pF  C-USC0603  [C0603]
R1  10k  R-US_R0402  [R0402]
R2  10k  R-US_R0402  [R0402]
R3  10k  R-US_R0402  [R0402]
R4  10k  R-US_R0402  [R0402]
R5  10k  R-US_R0402  [R0402]
R6  0  R-US_R0402  [R0402]
R7  0  R-US_R0402  [R0402]
R8  0  R-US_R0402  [R0402]
R10  0  R-US_R0402  [R0402]
R11  0  R-US_R0402  [R0402]
R12  5.6k  R-US_R0402  [R0402]
R13  5.6k  R-US_R0402  [R0402]
R14  5.6k  R-US_R0402  [R0402]
R15  0  R-US_R0402  [R0402]
R16  0  R-US_R0402  [R0402]
R28  5.6k  R-US_R0402  [R0402]
R29  10k  R-US_R0402  [R0402]
R34  1M  R-US_R0603  [R0603]
R40  0  R-US_R0402  [R0402]
R50  2k  R-US_R0402  [R0402]
TP1  TPPAD1-13  [P1-13]
TP2  TPPAD1-13  [P1-13]
U3  TPD4S012_DRY_6  [DRY6]
U6  JTAG_ARM_10PIN  [CON_2X5_50MIL]
U20  TM4C123GH6PMI  [LQFP-64-PM]
U21  TC2050-NL-MCP-NL  [TC2030-MCP-NL]
U22  CON_USB_FCI_MICRO_B_10118194  [CON_USB_MICRO_B_FCI_10118194]
X1  TSW-107-02-S-D  [TSW-107-02-S-D]
Y2  16M  NX3225GA  [NDK3.2X2.5]

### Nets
!DEBUG_RESET_OUT: R16.2 U6.P10(!RESET) U20.P$23(PA6) X1.1
!EXTERNAL_DEBUG: R40.1 TP2.TP U20.P$24(PA7)
!TARGET_RESET: R16.1 X1.2 ; also sheet 2,3,5
+3V3: C10.1 C11.1 C12.1 C13.1 R3.2 R4.1 R5.1 U6.P1(VTARGET) U20.P$2(VDDA) U20.P$11(VDD0) U20.P$26(VDD1) U20.P$37(VBAT) U20.P$42(VDD2) U20.P$54(VDD3) U21.1(VTREF) ; also sheet 2,3,5
DEBUG_ACTIVE: TP1.TP U20.P$64(PD3)
DEBUG_PC0/TCK/SWCLK: R8.2 U6.P4(TCK) U20.P$19(PA2) U20.P$30(PF2) X1.9
DEBUG_PC1/TMS/SWDIO: R10.2 U6.P2(TMS) U20.P$20(PA3) U20.P$29(PF1) X1.7
DEBUG_PC2/TDI: R11.2 U6.P8(TDI) U20.P$22(PA5) X1.5
DEBUG_PC3/TDO/SWO: R15.2 U6.P6(TDO) U20.P$21(PA4) U20.P$53(PD6) X1.3
DEBUG_VBUS: R28.2 U3.6(VBUS) U22.P1(VBUS) ; also sheet 5
GND: C2.2 C5.2 C6.2 C7.2 C8.2 C9.2 C10.2 C11.2 C12.2 C13.2 C33.2 R12.2 R13.2 R14.2 R29.1 R34.1 U3.4(GND) U6.P5(GND) U6.P9(GND1) U20.P$3(GNDA) U20.P$12(GND0) U20.P$27(GND1) U20.P$32(!WAKE) U20.P$34(XOSC0) U20.P$35(GNDX) U20.P$39(GND2) U20.P$55(GND3) U21.3(GND) U21.5(NC) U21.9(!TRST) U22.P5(GND) ; also sheet 1,2,3,4,5
ICDI_RESET: C2.1 R3.1 U20.P$38(!RESET) U21.10(RESET)
ICDI_TCK: R4.2 U20.P$52(PC0/TCK) U21.4(TCK)
ICDI_TDI: U20.P$50(PC2/TDI) U21.8(TDI)
ICDI_TDO: U20.P$49(PC3/TDO) U21.6(TDO)
ICDI_TMS: R5.2 U20.P$51(PC1/TMS) U21.2(TMS)
ICDI_USBD_N [USB]: U3.2(D-) U20.P$43(PD4) U22.P2(DM)
ICDI_USBD_P [USB]: U3.1(D+) U20.P$44(PD5) U22.P3(DP)
ICDI_VDDC: C5.1 C6.1 C7.1 U20.P$25(VDDC0) U20.P$56(VDDC1)
MCU_3V3: R1.1 R2.1 ; also sheet 4,5
N$1: C9.1 U20.P$40(OSC0) Y2.P$1(OSC0)
N$2: C8.1 R50.2 Y2.P$3(OSC1)
N$12: R40.2 U6.P3(!EXTDBG)
N$15: R28.1 R29.2 U20.P$46(PB1)
N$17: R50.1 U20.P$41(OSC1)
N$20: C33.1 R34.2 U22.P6(S1) U22.P7(S2) U22.P8(S3) U22.P9(S4) U22.P10(S5) U22.P11(S6)
TARGET_RXD: R7.1 X1.12 ; also sheet 2
TARGET_TCK/SWCLK: R1.2 R8.1 X1.10 ; also sheet 1
TARGET_TDI: R11.1 X1.6 ; also sheet 1
TARGET_TDO/SWO: R15.1 X1.4 ; also sheet 1
TARGET_TMS/SWDIO: R2.2 R10.1 X1.8 ; also sheet 1
TARGET_TXD: R6.1 X1.14 ; also sheet 2
VCP_RXD: R6.2 U20.P$17(PA0) X1.13
VCP_TXD: R7.2 U20.P$18(PA1) X1.11
VERSION_0: R12.1 U20.P$61(PD0)
VERSION_1: R13.1 U20.P$47(PB2)
VERSION_2: R14.1 U20.P$48(PB3)
Unconnected: U3.3(ID) U3.5(N.C.) U6.P7 U20.P$1(PB6) U20.P$4(PB7) U20.P$5(PF4) U20.P$6(PE3) U20.P$7(PE2) U20.P$8(PE1) U20.P$9(PE0) U20.P$10(PD7) U20.P$13(PC7) U20.P$14(PC6) U20.P$15(PC5) U20.P$16(PC4) U20.P$28(PF0) U20.P$31(PF3) U20.P$33(!HIB) U20.P$36(XOSC1) U20.P$45(PB0) U20.P$57(PB5) U20.P$58(PB4) U20.P$59(PE4) U20.P$60(PE5) U20.P$62(PD1) U20.P$63(PD2) U21.7(RTCK) U22.P4(ID) Y2.P$2(NC2) Y2.P$4(NC4)

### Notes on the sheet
- JTAG PULL-UPS
- Use this for JTAG IN from external debugger.  See X1 
  jumpers for information about debug out to an 
  external target. 
  R40 must be removed for debug out.
  R40 must be instaled for debug in.
- EXTERNAL_DEBUG pull low to use external debugger
  to debug the target.  Causes ICDI chip to tri-state the JTAG lines
- PE4 ETM_ENn Leave Open 
  use GPIO Internal weak pullup.
- PE5 LS_PRESENTn Leave Open
  use GPIO internal weak pullup
- VERSION RESISTOR TABLE:
  *use internal GPIO weak pullups.
  ALL OMITTED: Legacy mode. (Stellaris ICDI)
  ALL POPULATED: Everything enabled
  Version 0 populated: UART CTS/RTS and Analog inputs
- Jumpers to bridge from ICDI to Target portion of LaunchPad
- X1 omitted by default
  
  To debug out from ICDI to off board MCU remove 
  0 ohm jumper resistors.  To go back from debug 
  out to debugging the target MCU install X1 and 
  place jumpers on all pins.

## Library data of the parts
C1 = EK-TM4C1294XL REV A:C-US: CAPACITOR, American symbol; GNUM: G10-C1210-C102-ZCA
C2 = ek-tm4c129exl:C-US: CAPACITOR, American symbol; GNUM: G10-C0402-C104-HBA; POPOP: OMIT
C3-C5 C10-C13 C16-C19 C21-C30 C40-C43 C46 = ek-tm4c129exl:C-US: CAPACITOR, American symbol; GNUM: G10-C0402-C104-HBA
C6 C14 = ek-tm4c129exl:C-US: CAPACITOR, American symbol; GNUM: G10-C0402-C105-GBB
C7 = ek-tm4c129exl:C-US: CAPACITOR, American symbol; GNUM: G10-C0603-C225-HBB
C8 C9 C44 C45 C47 C48 = ek-tm4c129exl:C-US: CAPACITOR, American symbol; GNUM: G10-C0402-C120-AAC
C15 C20 = ek-tm4c129exl:C-US: CAPACITOR, American symbol; DIGIKEY_PARTNUM: 311-1451-2-ND; GNUM: G10-C0603-C225-HBB
C31 = ek-tm4c129exl:C-US: CAPACITOR, American symbol; GNUM: G10-C1812-C472-ZBA
C32 C33 = EK-TM4C1294XL REV A:C-US: CAPACITOR, American symbol; GNUM: G10-C0603-C332-ABA
D0 D1-D4 = ek-tm4c129exl:LED: LED; GNUM: G14-D0603-GR00-AAA
H1 H4 H6 = holes:MOUNT-HOLE: MOUNTING HOLE with drill center marker; GNUM: G30-62S04-A112-AAA; POPOP: OMIT
J1-J7 = jumper:JUMPER: JUMPER header; GNUM: G72-100MI-JMPA-AAA
JP1 = pinhead:PINHD-2X3: PIN HEADER; GNUM: G22-THVEU-2X3P-BAB
JP2 JP3 = pinhead:PINHD-1X2: PIN HEADER; GNUM: G22-THVEU-002P-AAA
JP4 JP5 = pinhead:PINHD-2X2: PIN HEADER; GNUM: G22-THVEU-002P-BAB
R1-R5 R29 R35 R44 = ek-tm4c129exl:R-US_: RESISTOR, American symbol; GNUM: G11-R0402-1002-AAA
R6-R8 R10 R11 R15 R16 R19 R20 R39-R41 = ek-tm4c129exl:R-US_: RESISTOR, American symbol; GNUM: G11-R0402-0000-AAA
R9 R27 R30 R31 R33 = ek-tm4c129exl:R-US_: RESISTOR, American symbol; GNUM: G11-R0402-3300-AAA
R12-R14 = ek-tm4c129exl:R-US_: RESISTOR, American symbol; GNUM: G11-R0402-5601-AAA; POPOP: OMIT
R17 R26 R36 = ek-tm4c129exl:R-US_: RESISTOR, American symbol; GNUM: G11-R0402-1003-AAA
R18 R51 = ek-tm4c129exl:R-US_: RESISTOR, American symbol; GNUM: G11-R0402-1000-AAA
R21-R24 = ek-tm4c129exl:R-US_: RESISTOR, American symbol; GNUM: G11-R0402-49R9-ABA
R25 = ek-tm4c129exl:R-US_: RESISTOR, American symbol; GNUM: G11-R0402-4871-ABA
R28 = ek-tm4c129exl:R-US_: RESISTOR, American symbol; GNUM: G11-R0402-5601-AAA
R32 R43 R45 R46 = ek-tm4c129exl:R-US_: RESISTOR, American symbol; GNUM: G11-R0402-75R0-AAA
R34 R52 = EK-TM4C1294XL REV A:R-US_: RESISTOR, American symbol; GNUM: G11-R0603-R105-AAA
R38 = ek-tm4c129exl:R-US_: RESISTOR, American symbol; GNUM: G11-R0402-51R0-AAA
R42 = ek-tm4c129exl:R-US_: RESISTOR, American symbol; GNUM: G11-R0402-1004-AAA
R47 = EK-TM4C1294XL REV A:R-US_: RESISTOR, American symbol; GNUM: G11-R1206-R105-CAA
R48 = ek-tm4c129exl:R-US_: RESISTOR, American symbol; GNUM: G11-R0402-5232-ABA; POPOP: OMIT
R49 R50 = ek-tm4c129exl:R-US_: RESISTOR, American symbol; GNUM: G11-R0402-R202-AAA
RESET USR_SW1 USR_SW2 WAKE = ek-tm4c129exl:SWITCH_TACTILE; GNUM: G21-4P6MM-B3S1-AAA
TP1-TP17 = ek-tm4c129exl:TP: Test pad; GNUM: G20-K5000-TP00-AAA; POPOP: OMIT
U1 = EK-TM4C1294XL REV A:TM4C1294NCPDT; GNUM: G50-QF128-C1294-ALH
U2 U3 = ek-tm4c129exl:TPD4S012_DRY_6; DATASHEETURL: http://www.ti.com/lit/gpn/TPD4S012; DESCRIPTION: 4-Channel USB ESD Solution with Power Clamp; FAMILY_NAME: ESD Solution; GENERIC_PART_NUMBER: TPD4S012; GNUM: G57-SMDRY-S012-AAA; INDUSTRY_STD_PKG_TYPE: SON; MANUFACTURER: Texas Instruments; MANUFACTURER_PART_NUMBER: tpd4s012_dry_6; PACKAGE_DESIGNATOR: DRY; PIN_COUNT: 6; VENDOR: Texas Instruments
U4 = ek-tm4c129exl:TPS2052B_DRB_8; DATASHEETURL: http://www.ti.com/lit/gpn/TPS2052B; DESCRIPTION: Current-Limited, Power-Distribution Switches; FAMILY_NAME: USB POWER SWITCH; GENERIC_PART_NUMBER: TPS2052B; GNUM: G57-08SON-2052-AAA; INDUSTRY_STD_PKG_TYPE: SON; MANUFACTURER: Texas Instruments; MANUFACTURER_PART_NUMBER: tps2052b_drb_8; PACKAGE_DESIGNATOR: DRB; PIN_COUNT: 8; VENDOR: Texas Instruments
U5 = ek-tm4c129exl:TPS73733_DRV_6; GNUM: G51-DRV06-T733-AAA
U6 = ek-tm4c129exl:JTAG_ARM_10PIN; GNUM: G22-SMVES-2X5A-BBC
U7 = ek-tm4c129exl:CON_USB_HIROSE_MICRO_AB_ZX62D_AB_5P8; GNUM: G20-USBU-THAB-CEB
U8 U9 = SparkFun-DigitalIC:ATMEGA328P_PDIP: uC used in the Arduino 32kb flash, 1k EEPROM, 2k SRAM This is the through-hole version of this chip.
U10 = ek-tm4c129exl:MAG_PULSE_HX1188FNL; GNUM: G12-SOI16-1TO1-ZZQ
U11 = SerialPortBluetooth:HC_05
U13 = ek-tm4c129exl:SLVU2.8-4; GNUM: G14-SOIC8-SLVU-DAA
U14 = ek-tm4c129exl:JACK_RJ45_NOMAG_NOLED_TECON; GNUM: G20-8RJ45-ENET-AAA
U20 = ek-tm4c129exl:TM4C123GH6PMI; GNUM: G50-QFP64-F120-EGC
U21 = ek-tm4c129exl:TC2050-NL: TAG-CONNECT ISP Connector Manufacturer: Tag-Connect Cable for easy In-Circuit PCB Programming. Designed for JTAG 10 pin, suitable for many others. Pin Connection for TC2050 NL. PADDescription 1VTREF 2TMS 3GND 4TCK 5NC 6TDO 7RTCK 8TDI 9!TRST 10RESET ©2009 ROFA.cz Modified 7/2011 by Tim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; POPOP: OMIT
U22 = ek-tm4c129exl:CON_USB_FCI_MICRO_B_10118194; GNUM: G20-USBU-THB-CEB
X1 = ek-tm4c129exl:TSW-107-02-S-D: THROUGH-HOLE .025" SQ POST HEADER Source: Samtec TSW.pdf; GNUM: G22-THVEU-2X7P-BAB; OC_FARNELL: unknown; OC_NEWARK: unknown; POPOP: OMIT
X6-X9 = ek-tm4c129exl:TSW-110-02-S-D: THROUGH-HOLE .025" SQ POST HEADER Source: Samtec TSW.pdf; GNUM: G22-THSTK-2X10-BAC; OC_FARNELL: unknown; OC_NEWARK: unknown
X11 = con-samtec:TSW-149-02-S-D: THROUGH-HOLE .025" SQ POST HEADER Source: Samtec TSW.pdf; GNUM1: G22-THRE-1x49-AAC; GNUM2: G22-THRA-1X49-AAC; OC_FARNELL: unknown; OC_NEWARK: unknown; POPOP: OMIT
Y1 = ek-tm4c129exl:NX3225GA; GNUM: G15-32X25-2506-AAA
Y2 = ek-tm4c129exl:NX3225GA; GNUM: G15-32X25-1606-AAA
Y3 = EK-TM4C1294XL REV A:CRYATL_32K_SMD; GNUM: G15-CMR2T-3272-AAA

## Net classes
1 USB: width 0.275 mm, clearance 0.152 mm
2 Ethernet: width 0.22 mm, clearance 0.152 mm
